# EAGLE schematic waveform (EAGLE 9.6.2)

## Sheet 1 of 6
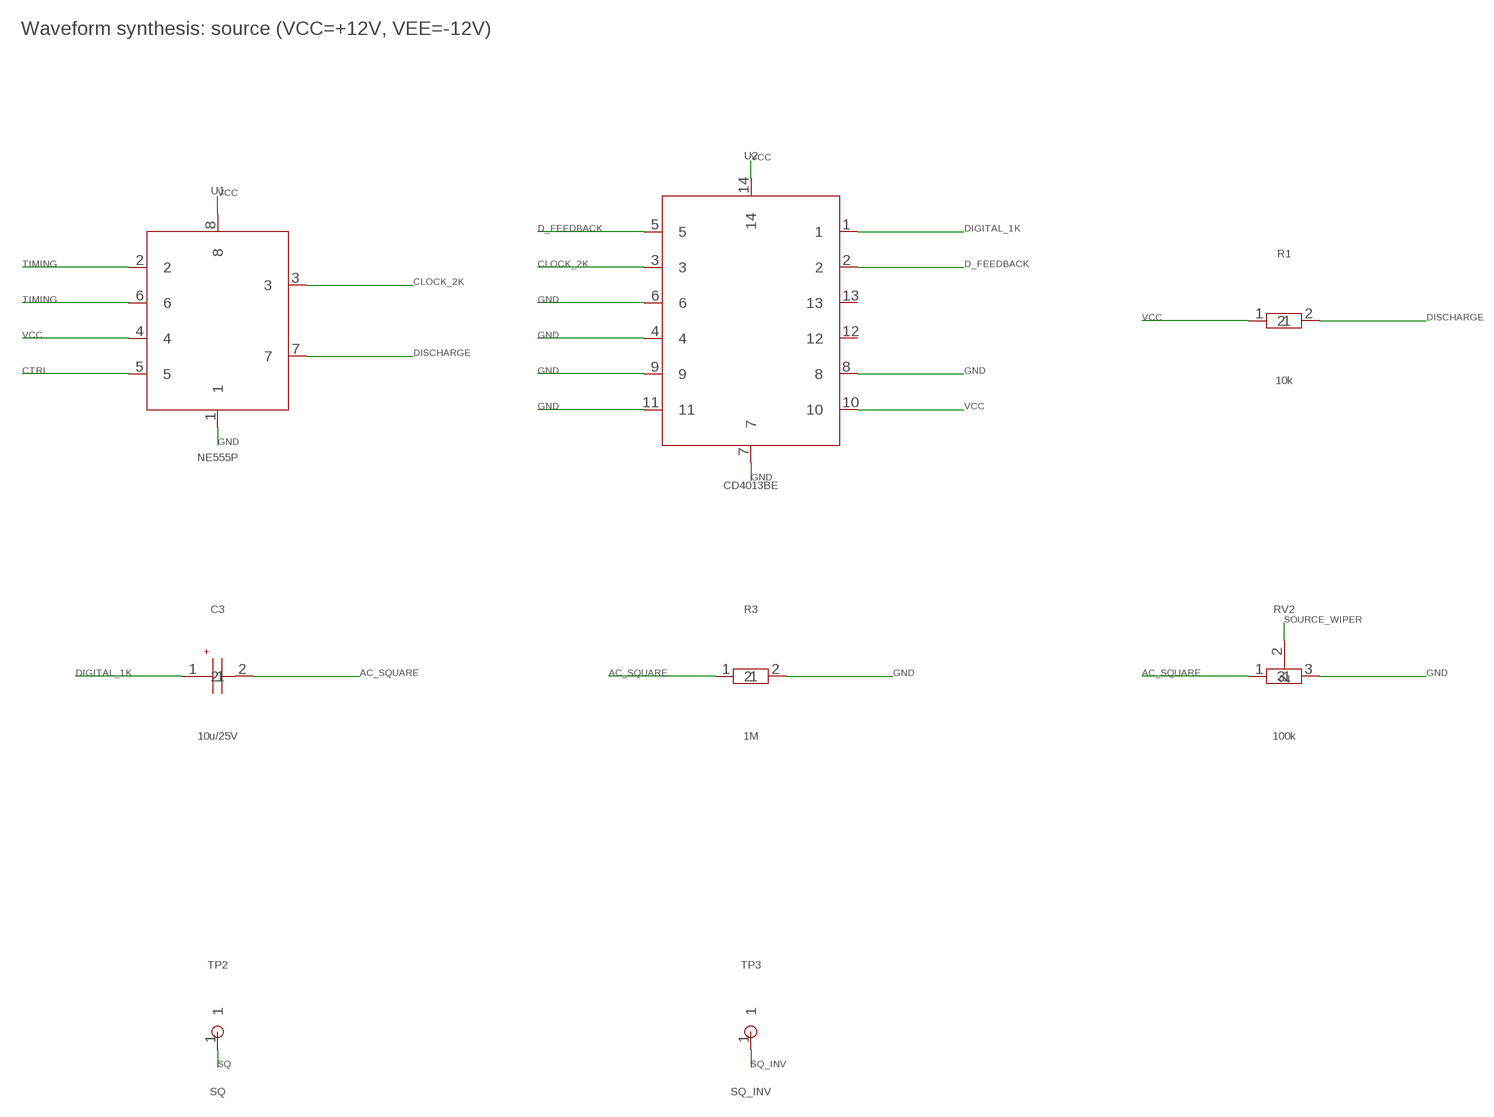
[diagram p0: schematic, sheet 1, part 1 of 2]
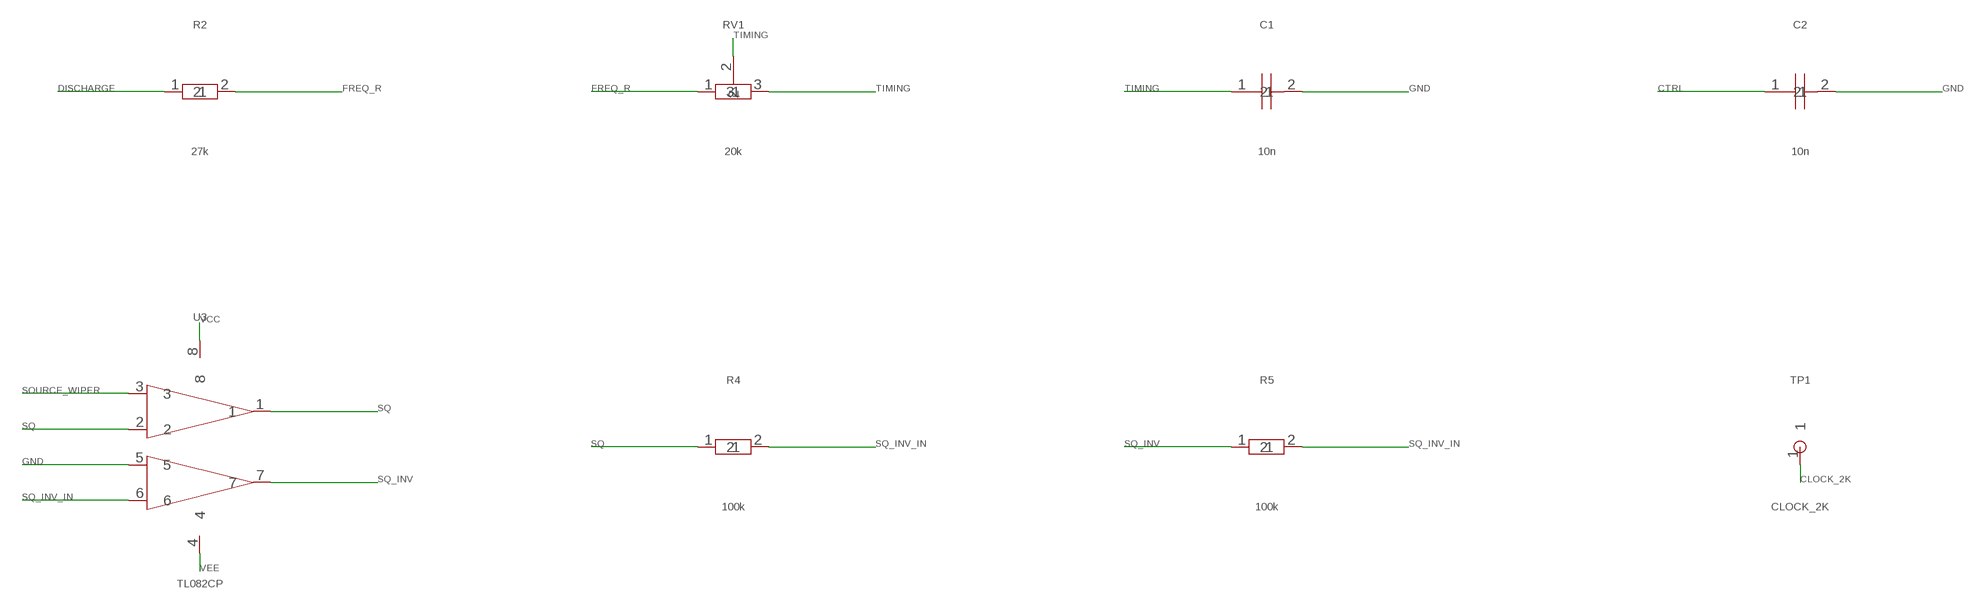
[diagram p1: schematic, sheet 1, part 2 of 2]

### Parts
C1  10n  C  [C_Disc_D5.0mm_W2.5mm_P5.00mm]
C2  10n  C  [C_Disc_D5.0mm_W2.5mm_P5.00mm]
C3  10u/25V  CP  [CP_Radial_D5.0mm_P2.00mm]
R1  10k  R  [R_Axial_DIN0207_L6.3mm_D2.5mm_P7.62mm_Horizontal]
R2  27k  R  [R_Axial_DIN0207_L6.3mm_D2.5mm_P7.62mm_Horizontal]
R3  1M  R  [R_Axial_DIN0207_L6.3mm_D2.5mm_P7.62mm_Horizontal]
R4  100k  R  [R_Axial_DIN0207_L6.3mm_D2.5mm_P7.62mm_Horizontal]
R5  100k  R  [R_Axial_DIN0207_L6.3mm_D2.5mm_P7.62mm_Horizontal]
RV1  20k  POT  [Potentiometer_Bourns_3296W_Vertical]
RV2  100k  POT  [Potentiometer_Bourns_3296W_Vertical]
TP1  CLOCK_2K  TP  [TestPoint_THTPad_D1.5mm_Drill0.7mm]
TP2  SQ  TP  [TestPoint_THTPad_D1.5mm_Drill0.7mm]
TP3  SQ_INV  TP  [TestPoint_THTPad_D1.5mm_Drill0.7mm]
U1  NE555P  NE555  [DIP-8_W7.62mm]
U2  CD4013BE  4013  [DIP-14_W7.62mm]
U3  TL082CP  TL082  [DIP-8_W7.62mm]

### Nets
AC_SQUARE: C3.2 R3.1 RV2.1
CLOCK_2K: TP1.1 U1.3 U2.3
CTRL: C2.1 U1.5
D_FEEDBACK: U2.2 U2.5
DIGITAL_1K: C3.1 U2.1
DISCHARGE: R1.2 R2.1 U1.7
FREQ_R: R2.2 RV1.1
GND: C1.2 C2.2 R3.2 RV2.3 U1.1 U2.4 U2.6 U2.7 U2.8 U2.9 U2.11 U3.5 ; also sheet 2,3,4,5,6
SOURCE_WIPER: RV2.2 U3.3
SQ: R4.1 TP2.1 U3.1 U3.2 ; also sheet 2,3,4,5
SQ_INV: R5.1 TP3.1 U3.7
SQ_INV_IN: R4.2 R5.2 U3.6
TIMING: C1.1 RV1.2 RV1.3 U1.2 U1.6
VCC: R1.1 U1.4 U1.8 U2.10 U2.14 U3.8 ; also sheet 2,3,4,5,6
VEE: U3.4 ; also sheet 2,3,4,5,6
Unconnected: U2.12 U2.13

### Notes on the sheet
- Waveform synthesis: source (VCC=+12V, VEE=-12V)

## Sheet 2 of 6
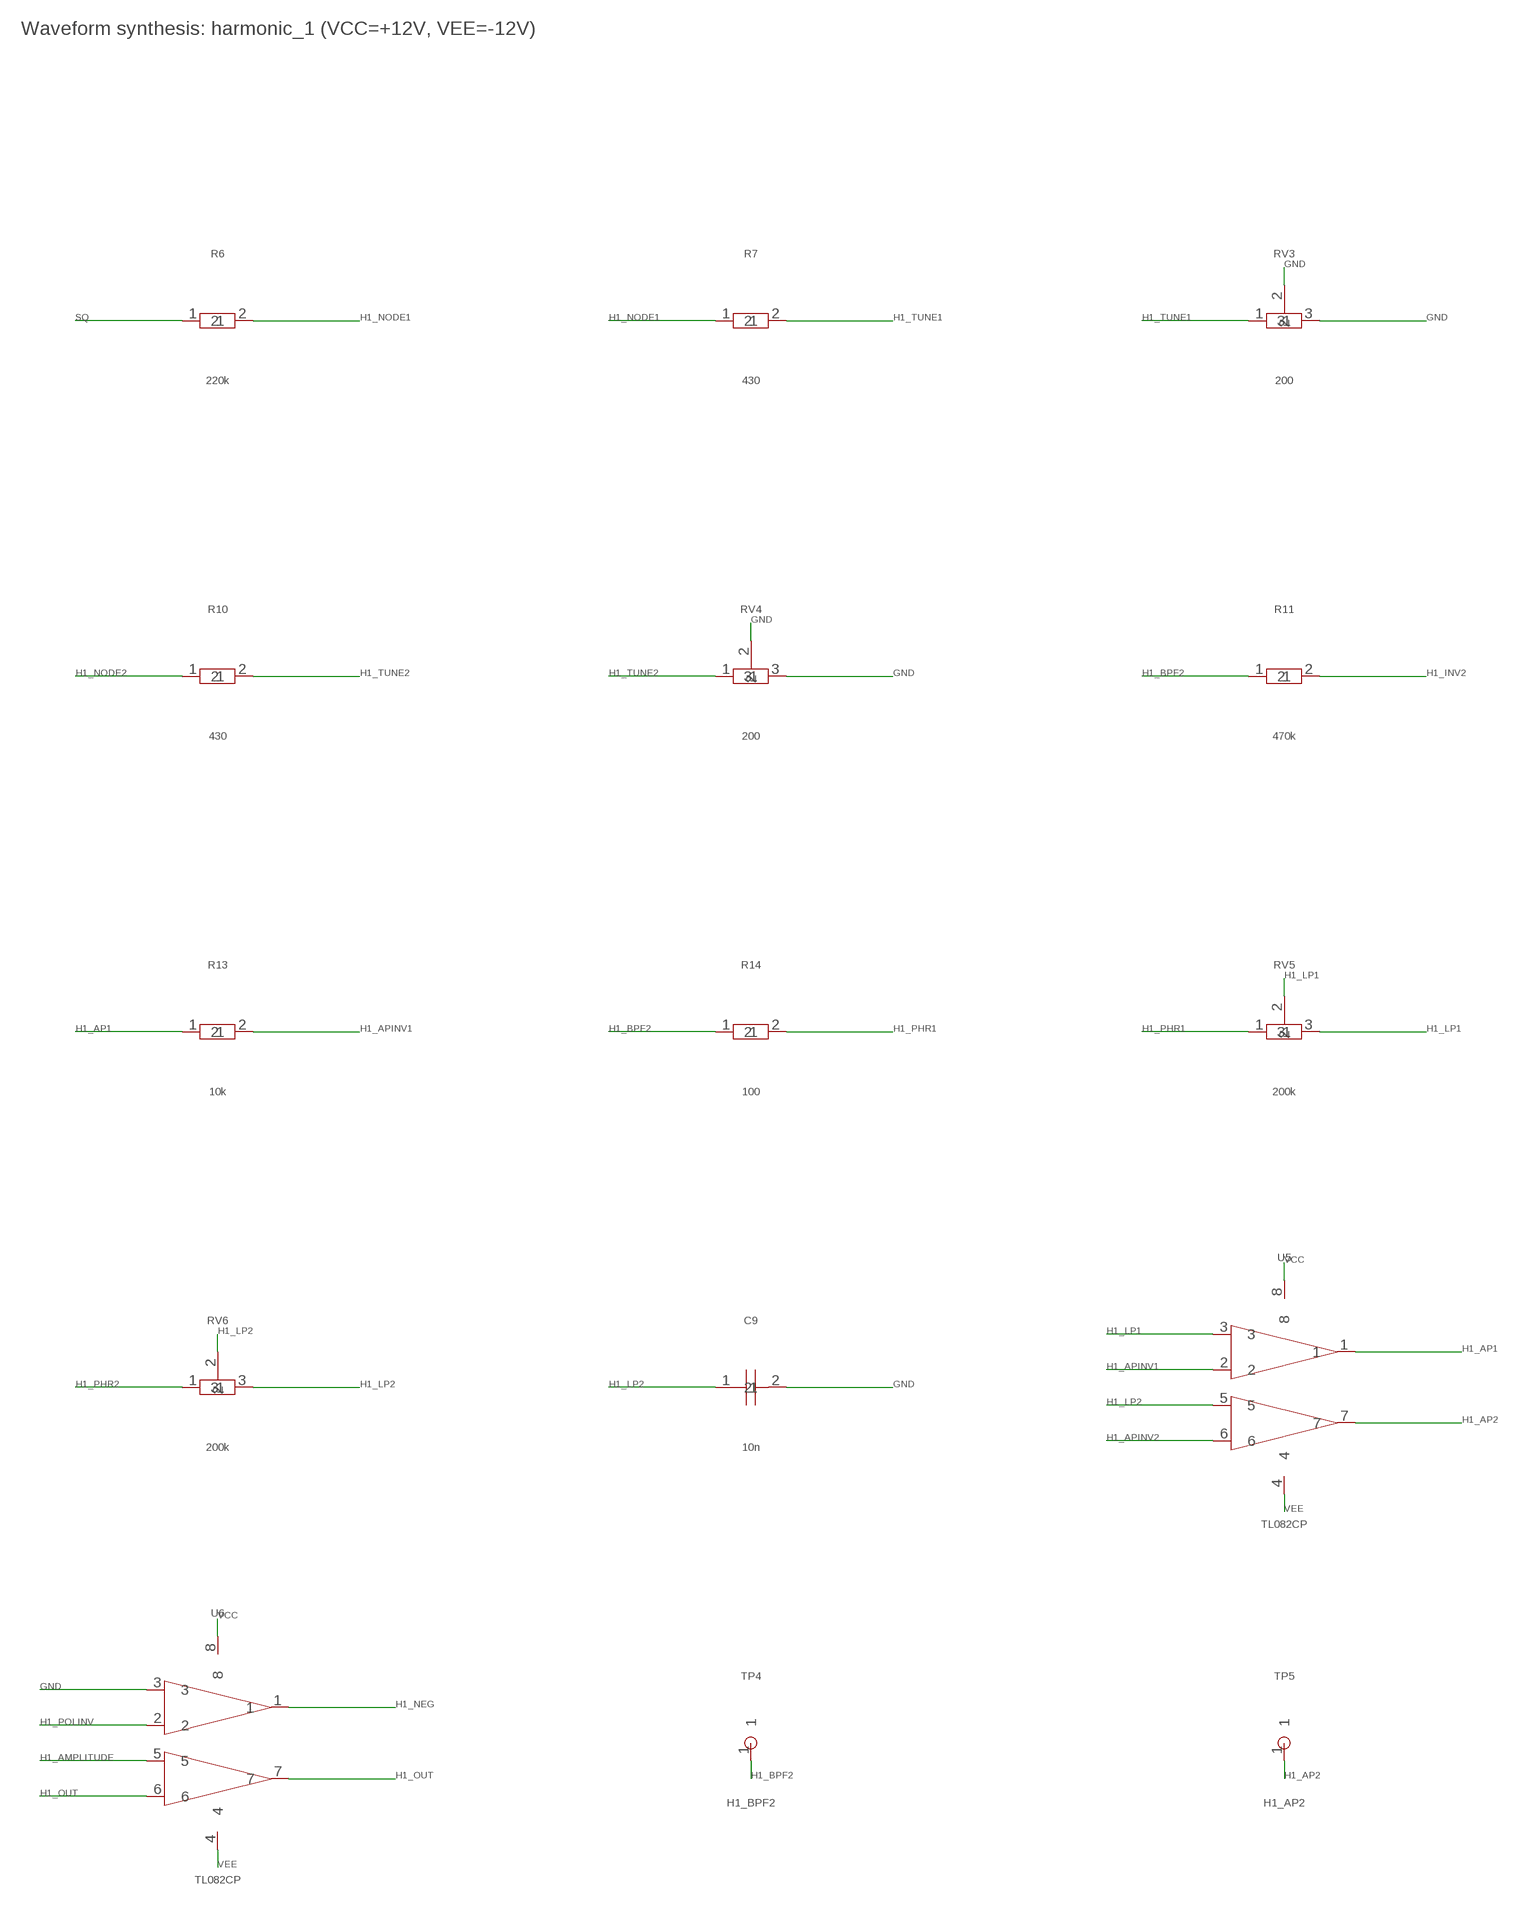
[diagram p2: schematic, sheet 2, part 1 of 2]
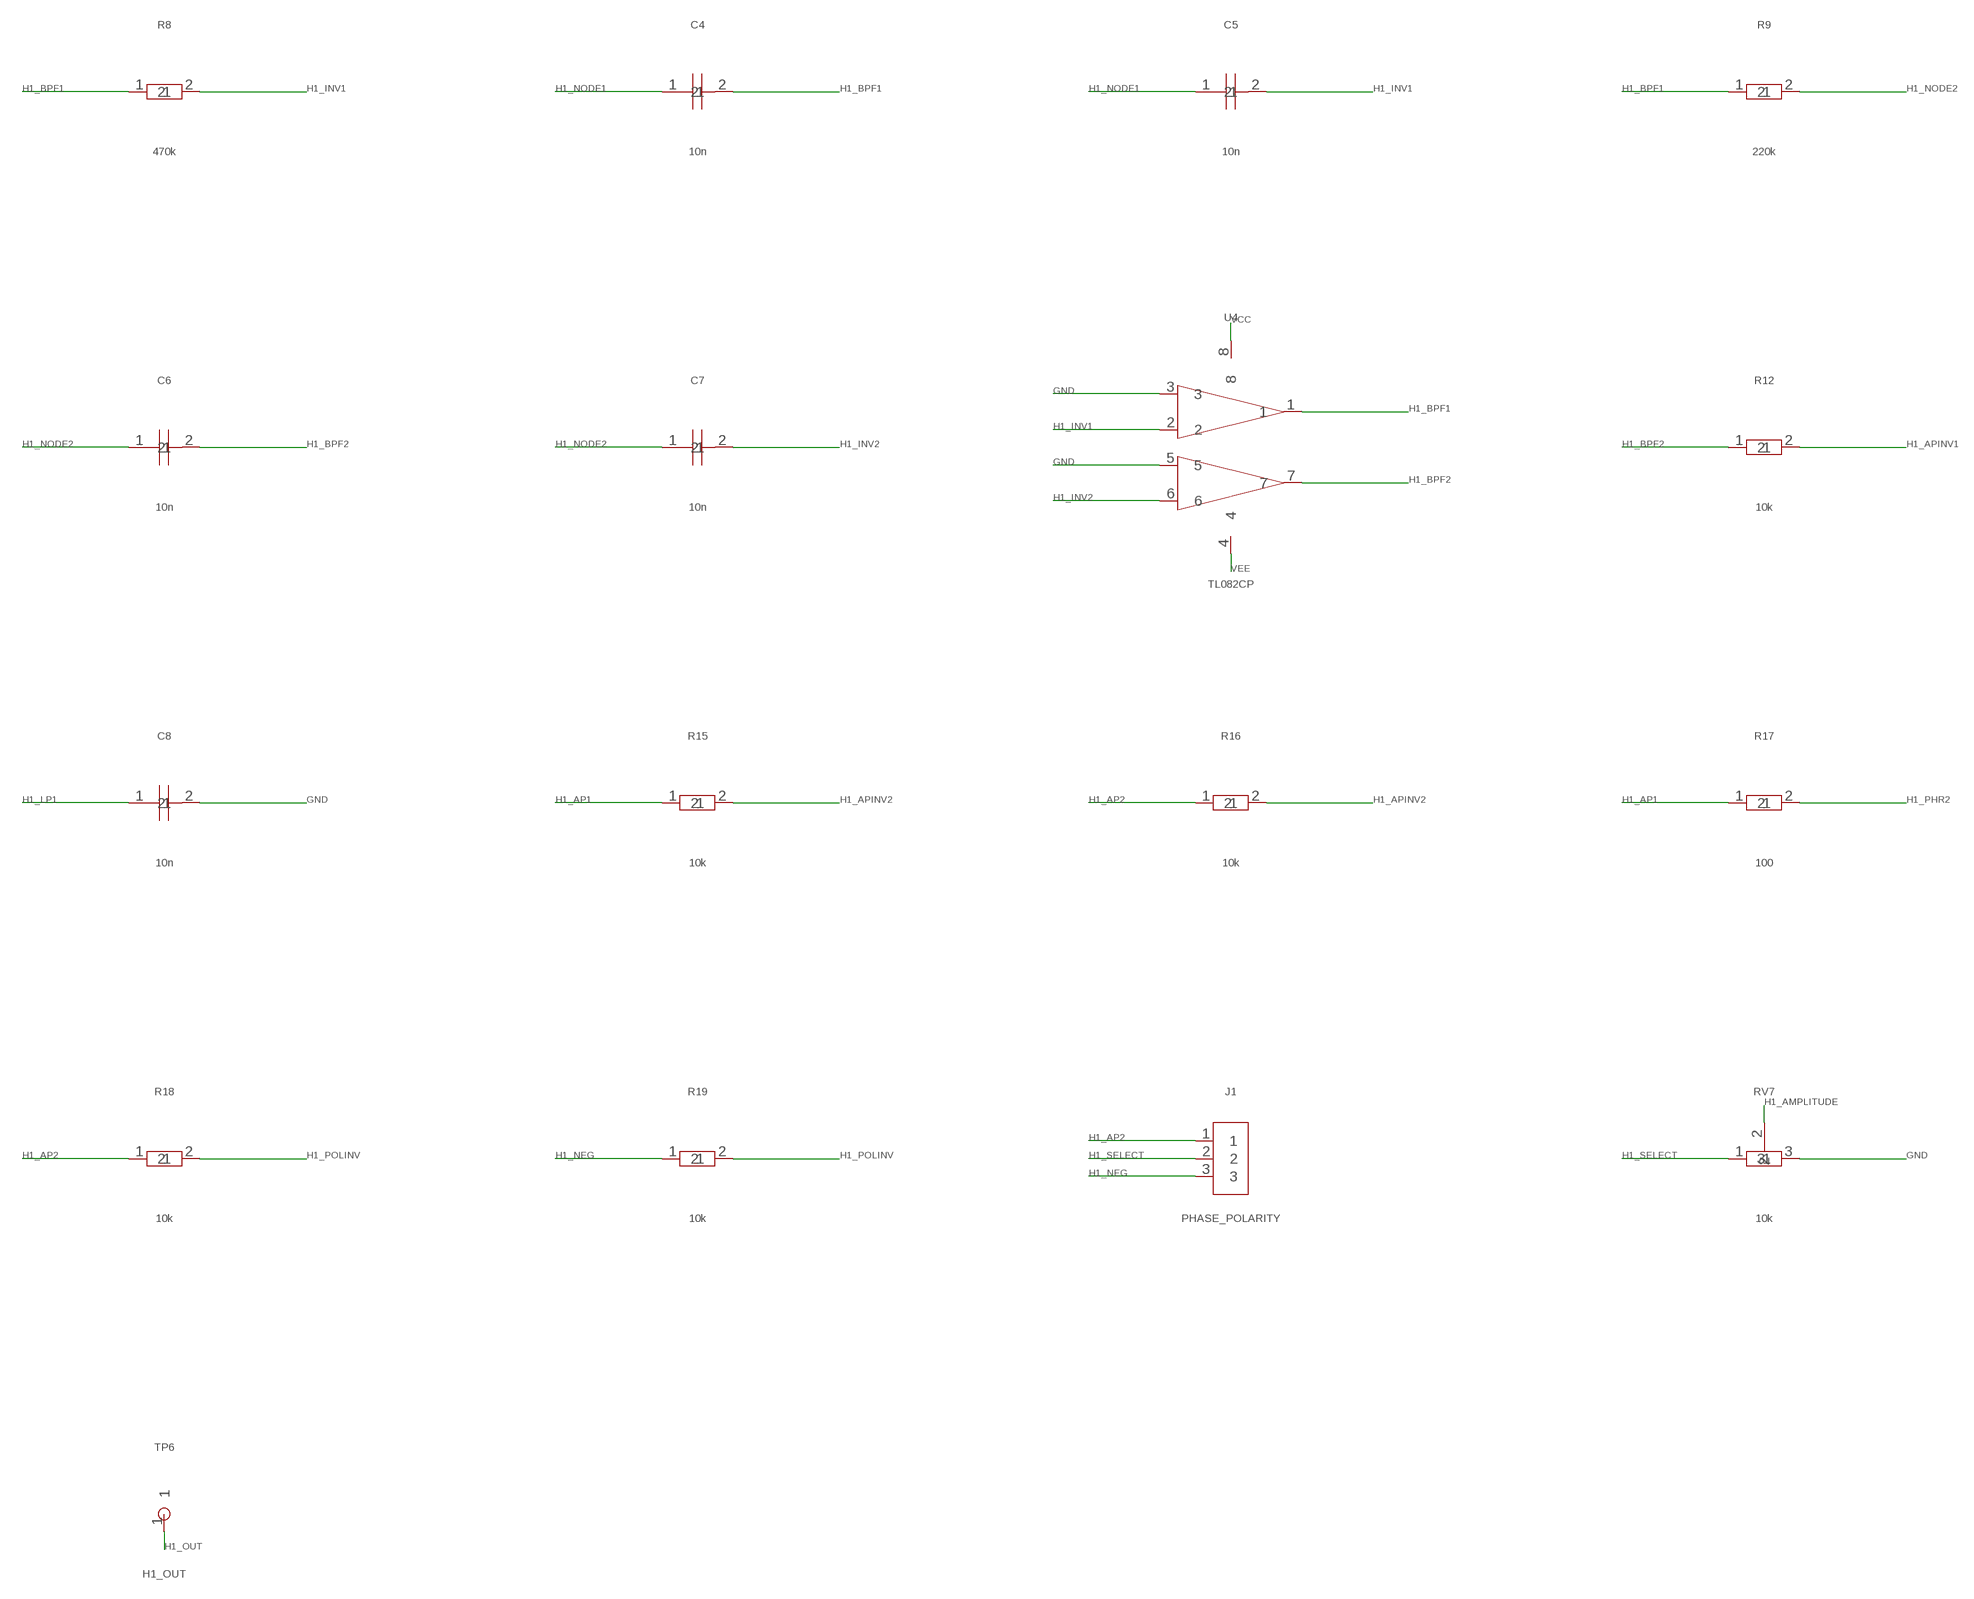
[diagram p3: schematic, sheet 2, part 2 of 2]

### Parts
C4  10n  C  [C_Disc_D5.0mm_W2.5mm_P5.00mm]
C5  10n  C  [C_Disc_D5.0mm_W2.5mm_P5.00mm]
C6  10n  C  [C_Disc_D5.0mm_W2.5mm_P5.00mm]
C7  10n  C  [C_Disc_D5.0mm_W2.5mm_P5.00mm]
C8  10n  C  [C_Disc_D5.0mm_W2.5mm_P5.00mm]
C9  10n  C  [C_Disc_D5.0mm_W2.5mm_P5.00mm]
J1  PHASE_POLARITY  CONN3  [PinHeader_1x03_P2.54mm_Vertical]
R6  220k  R  [R_Axial_DIN0207_L6.3mm_D2.5mm_P7.62mm_Horizontal]
R7  430  R  [R_Axial_DIN0207_L6.3mm_D2.5mm_P7.62mm_Horizontal]
R8  470k  R  [R_Axial_DIN0207_L6.3mm_D2.5mm_P7.62mm_Horizontal]
R9  220k  R  [R_Axial_DIN0207_L6.3mm_D2.5mm_P7.62mm_Horizontal]
R10  430  R  [R_Axial_DIN0207_L6.3mm_D2.5mm_P7.62mm_Horizontal]
R11  470k  R  [R_Axial_DIN0207_L6.3mm_D2.5mm_P7.62mm_Horizontal]
R12  10k  R  [R_Axial_DIN0207_L6.3mm_D2.5mm_P7.62mm_Horizontal]
R13  10k  R  [R_Axial_DIN0207_L6.3mm_D2.5mm_P7.62mm_Horizontal]
R14  100  R  [R_Axial_DIN0207_L6.3mm_D2.5mm_P7.62mm_Horizontal]
R15  10k  R  [R_Axial_DIN0207_L6.3mm_D2.5mm_P7.62mm_Horizontal]
R16  10k  R  [R_Axial_DIN0207_L6.3mm_D2.5mm_P7.62mm_Horizontal]
R17  100  R  [R_Axial_DIN0207_L6.3mm_D2.5mm_P7.62mm_Horizontal]
R18  10k  R  [R_Axial_DIN0207_L6.3mm_D2.5mm_P7.62mm_Horizontal]
R19  10k  R  [R_Axial_DIN0207_L6.3mm_D2.5mm_P7.62mm_Horizontal]
RV3  200  POT  [Potentiometer_Bourns_3296W_Vertical]
RV4  200  POT  [Potentiometer_Bourns_3296W_Vertical]
RV5  200k  POT  [Potentiometer_Bourns_3296W_Vertical]
RV6  200k  POT  [Potentiometer_Bourns_3296W_Vertical]
RV7  10k  POT  [Potentiometer_Bourns_3296W_Vertical]
TP4  H1_BPF2  TP  [TestPoint_THTPad_D1.5mm_Drill0.7mm]
TP5  H1_AP2  TP  [TestPoint_THTPad_D1.5mm_Drill0.7mm]
TP6  H1_OUT  TP  [TestPoint_THTPad_D1.5mm_Drill0.7mm]
U4  TL082CP  TL082  [DIP-8_W7.62mm]
U5  TL082CP  TL082  [DIP-8_W7.62mm]
U6  TL082CP  TL082  [DIP-8_W7.62mm]

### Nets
GND: C8.2 C9.2 RV3.2 RV3.3 RV4.2 RV4.3 RV7.3 U4.3 U4.5 U6.3 ; also sheet 1,3,4,5,6
H1_AMPLITUDE: RV7.2 U6.5
H1_AP1: R13.1 R15.1 R17.1 U5.1
H1_AP2: J1.1 R16.1 R18.1 TP5.1 U5.7
H1_APINV1: R12.2 R13.2 U5.2
H1_APINV2: R15.2 R16.2 U5.6
H1_BPF1: C4.2 R8.1 R9.1 U4.1
H1_BPF2: C6.2 R11.1 R12.1 R14.1 TP4.1 U4.7
H1_INV1: C5.2 R8.2 U4.2
H1_INV2: C7.2 R11.2 U4.6
H1_LP1: C8.1 RV5.2 RV5.3 U5.3
H1_LP2: C9.1 RV6.2 RV6.3 U5.5
H1_NEG: J1.3 R19.1 U6.1
H1_NODE1: C4.1 C5.1 R6.2 R7.1
H1_NODE2: C6.1 C7.1 R9.2 R10.1
H1_OUT: TP6.1 U6.6 U6.7 ; also sheet 6
H1_PHR1: R14.2 RV5.1
H1_PHR2: R17.2 RV6.1
H1_POLINV: R18.2 R19.2 U6.2
H1_SELECT: J1.2 RV7.1
H1_TUNE1: R7.2 RV3.1
H1_TUNE2: R10.2 RV4.1
SQ: R6.1 ; also sheet 1,3,4,5
VCC: U4.8 U5.8 U6.8 ; also sheet 1,3,4,5,6
VEE: U4.4 U5.4 U6.4 ; also sheet 1,3,4,5,6

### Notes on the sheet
- Waveform synthesis: harmonic_1 (VCC=+12V, VEE=-12V)

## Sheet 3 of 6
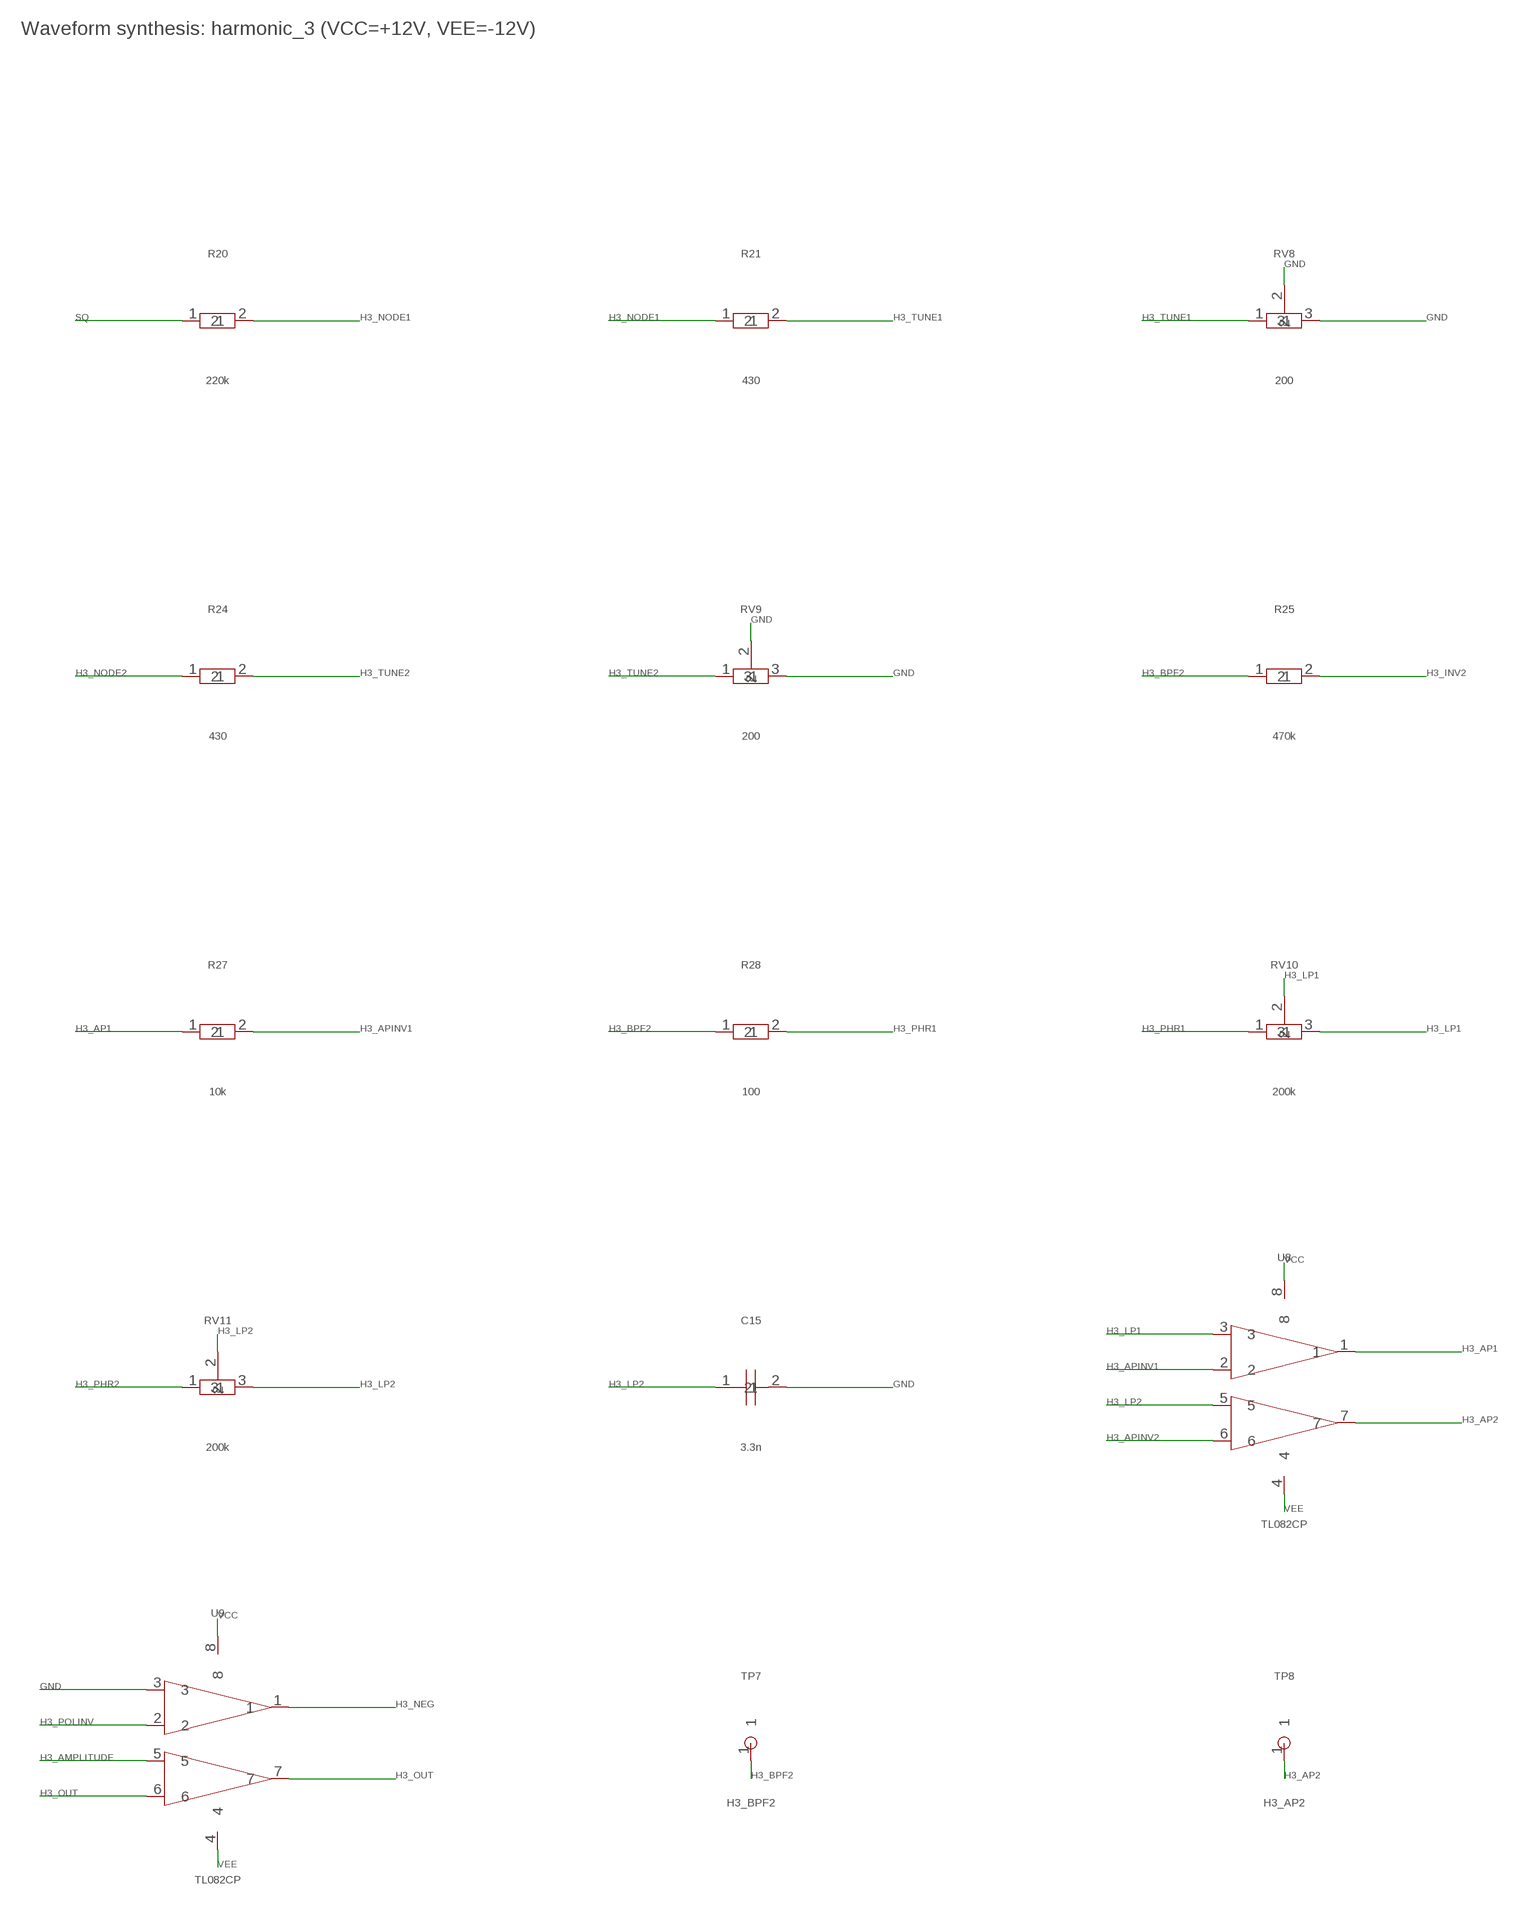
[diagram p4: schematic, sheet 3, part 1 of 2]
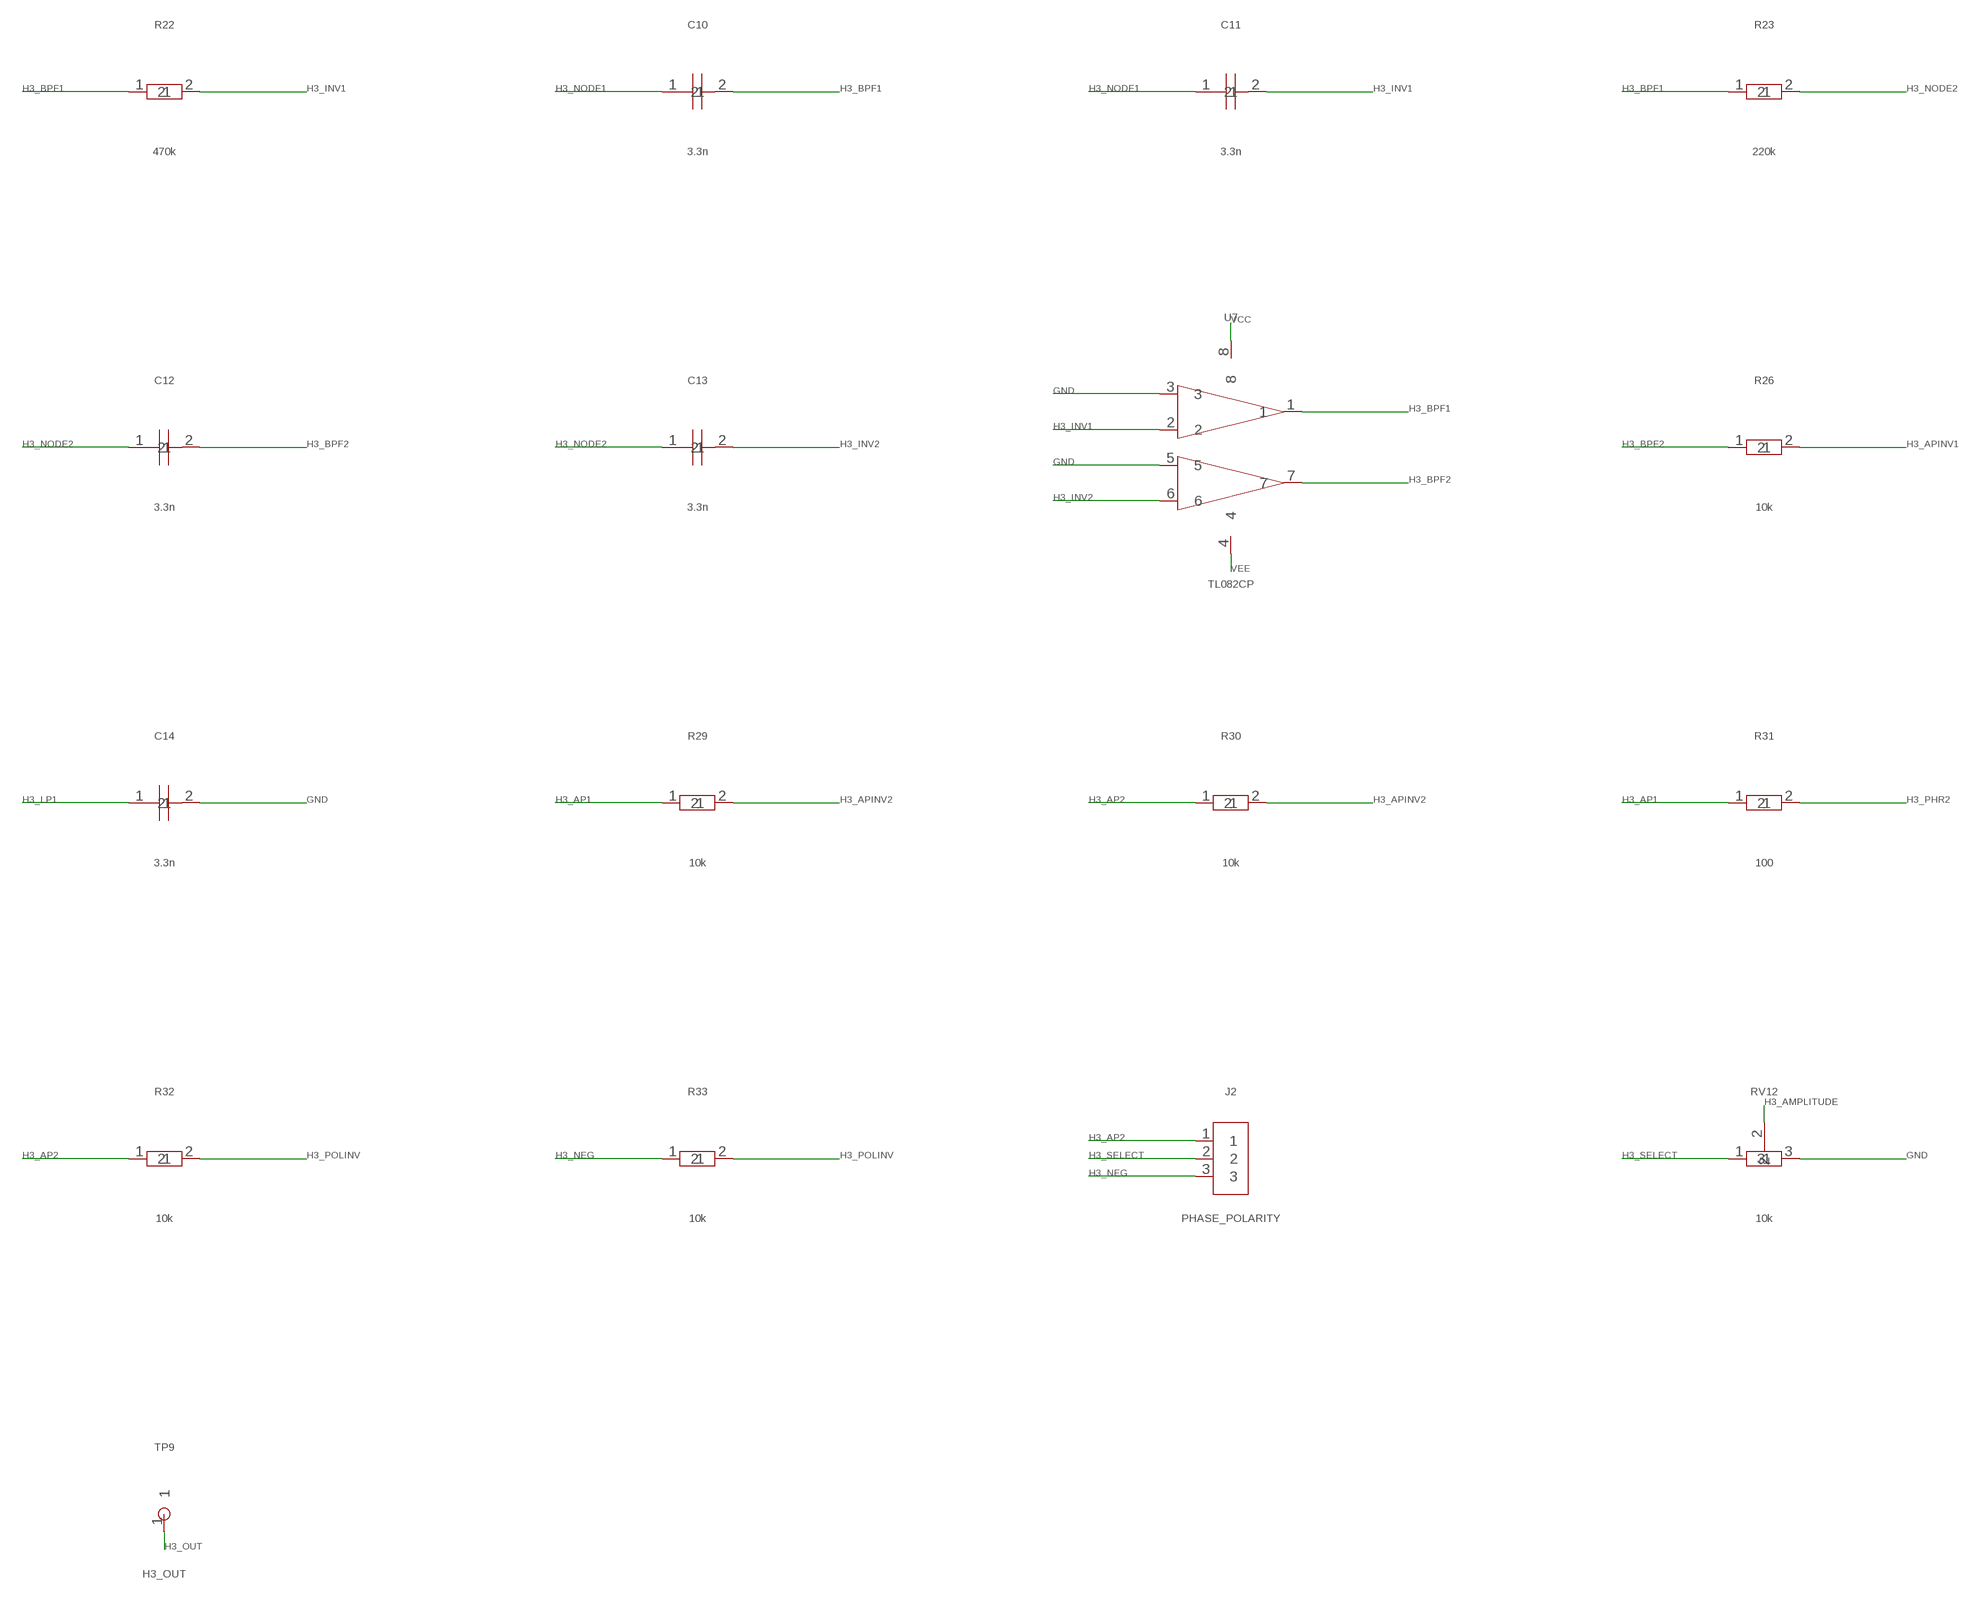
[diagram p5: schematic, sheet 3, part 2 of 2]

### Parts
C10  3.3n  C  [C_Disc_D5.0mm_W2.5mm_P5.00mm]
C11  3.3n  C  [C_Disc_D5.0mm_W2.5mm_P5.00mm]
C12  3.3n  C  [C_Disc_D5.0mm_W2.5mm_P5.00mm]
C13  3.3n  C  [C_Disc_D5.0mm_W2.5mm_P5.00mm]
C14  3.3n  C  [C_Disc_D5.0mm_W2.5mm_P5.00mm]
C15  3.3n  C  [C_Disc_D5.0mm_W2.5mm_P5.00mm]
J2  PHASE_POLARITY  CONN3  [PinHeader_1x03_P2.54mm_Vertical]
R20  220k  R  [R_Axial_DIN0207_L6.3mm_D2.5mm_P7.62mm_Horizontal]
R21  430  R  [R_Axial_DIN0207_L6.3mm_D2.5mm_P7.62mm_Horizontal]
R22  470k  R  [R_Axial_DIN0207_L6.3mm_D2.5mm_P7.62mm_Horizontal]
R23  220k  R  [R_Axial_DIN0207_L6.3mm_D2.5mm_P7.62mm_Horizontal]
R24  430  R  [R_Axial_DIN0207_L6.3mm_D2.5mm_P7.62mm_Horizontal]
R25  470k  R  [R_Axial_DIN0207_L6.3mm_D2.5mm_P7.62mm_Horizontal]
R26  10k  R  [R_Axial_DIN0207_L6.3mm_D2.5mm_P7.62mm_Horizontal]
R27  10k  R  [R_Axial_DIN0207_L6.3mm_D2.5mm_P7.62mm_Horizontal]
R28  100  R  [R_Axial_DIN0207_L6.3mm_D2.5mm_P7.62mm_Horizontal]
R29  10k  R  [R_Axial_DIN0207_L6.3mm_D2.5mm_P7.62mm_Horizontal]
R30  10k  R  [R_Axial_DIN0207_L6.3mm_D2.5mm_P7.62mm_Horizontal]
R31  100  R  [R_Axial_DIN0207_L6.3mm_D2.5mm_P7.62mm_Horizontal]
R32  10k  R  [R_Axial_DIN0207_L6.3mm_D2.5mm_P7.62mm_Horizontal]
R33  10k  R  [R_Axial_DIN0207_L6.3mm_D2.5mm_P7.62mm_Horizontal]
RV8  200  POT  [Potentiometer_Bourns_3296W_Vertical]
RV9  200  POT  [Potentiometer_Bourns_3296W_Vertical]
RV10  200k  POT  [Potentiometer_Bourns_3296W_Vertical]
RV11  200k  POT  [Potentiometer_Bourns_3296W_Vertical]
RV12  10k  POT  [Potentiometer_Bourns_3296W_Vertical]
TP7  H3_BPF2  TP  [TestPoint_THTPad_D1.5mm_Drill0.7mm]
TP8  H3_AP2  TP  [TestPoint_THTPad_D1.5mm_Drill0.7mm]
TP9  H3_OUT  TP  [TestPoint_THTPad_D1.5mm_Drill0.7mm]
U7  TL082CP  TL082  [DIP-8_W7.62mm]
U8  TL082CP  TL082  [DIP-8_W7.62mm]
U9  TL082CP  TL082  [DIP-8_W7.62mm]

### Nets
GND: C14.2 C15.2 RV8.2 RV8.3 RV9.2 RV9.3 RV12.3 U7.3 U7.5 U9.3 ; also sheet 1,2,4,5,6
H3_AMPLITUDE: RV12.2 U9.5
H3_AP1: R27.1 R29.1 R31.1 U8.1
H3_AP2: J2.1 R30.1 R32.1 TP8.1 U8.7
H3_APINV1: R26.2 R27.2 U8.2
H3_APINV2: R29.2 R30.2 U8.6
H3_BPF1: C10.2 R22.1 R23.1 U7.1
H3_BPF2: C12.2 R25.1 R26.1 R28.1 TP7.1 U7.7
H3_INV1: C11.2 R22.2 U7.2
H3_INV2: C13.2 R25.2 U7.6
H3_LP1: C14.1 RV10.2 RV10.3 U8.3
H3_LP2: C15.1 RV11.2 RV11.3 U8.5
H3_NEG: J2.3 R33.1 U9.1
H3_NODE1: C10.1 C11.1 R20.2 R21.1
H3_NODE2: C12.1 C13.1 R23.2 R24.1
H3_OUT: TP9.1 U9.6 U9.7 ; also sheet 6
H3_PHR1: R28.2 RV10.1
H3_PHR2: R31.2 RV11.1
H3_POLINV: R32.2 R33.2 U9.2
H3_SELECT: J2.2 RV12.1
H3_TUNE1: R21.2 RV8.1
H3_TUNE2: R24.2 RV9.1
SQ: R20.1 ; also sheet 1,2,4,5
VCC: U7.8 U8.8 U9.8 ; also sheet 1,2,4,5,6
VEE: U7.4 U8.4 U9.4 ; also sheet 1,2,4,5,6

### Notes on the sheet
- Waveform synthesis: harmonic_3 (VCC=+12V, VEE=-12V)

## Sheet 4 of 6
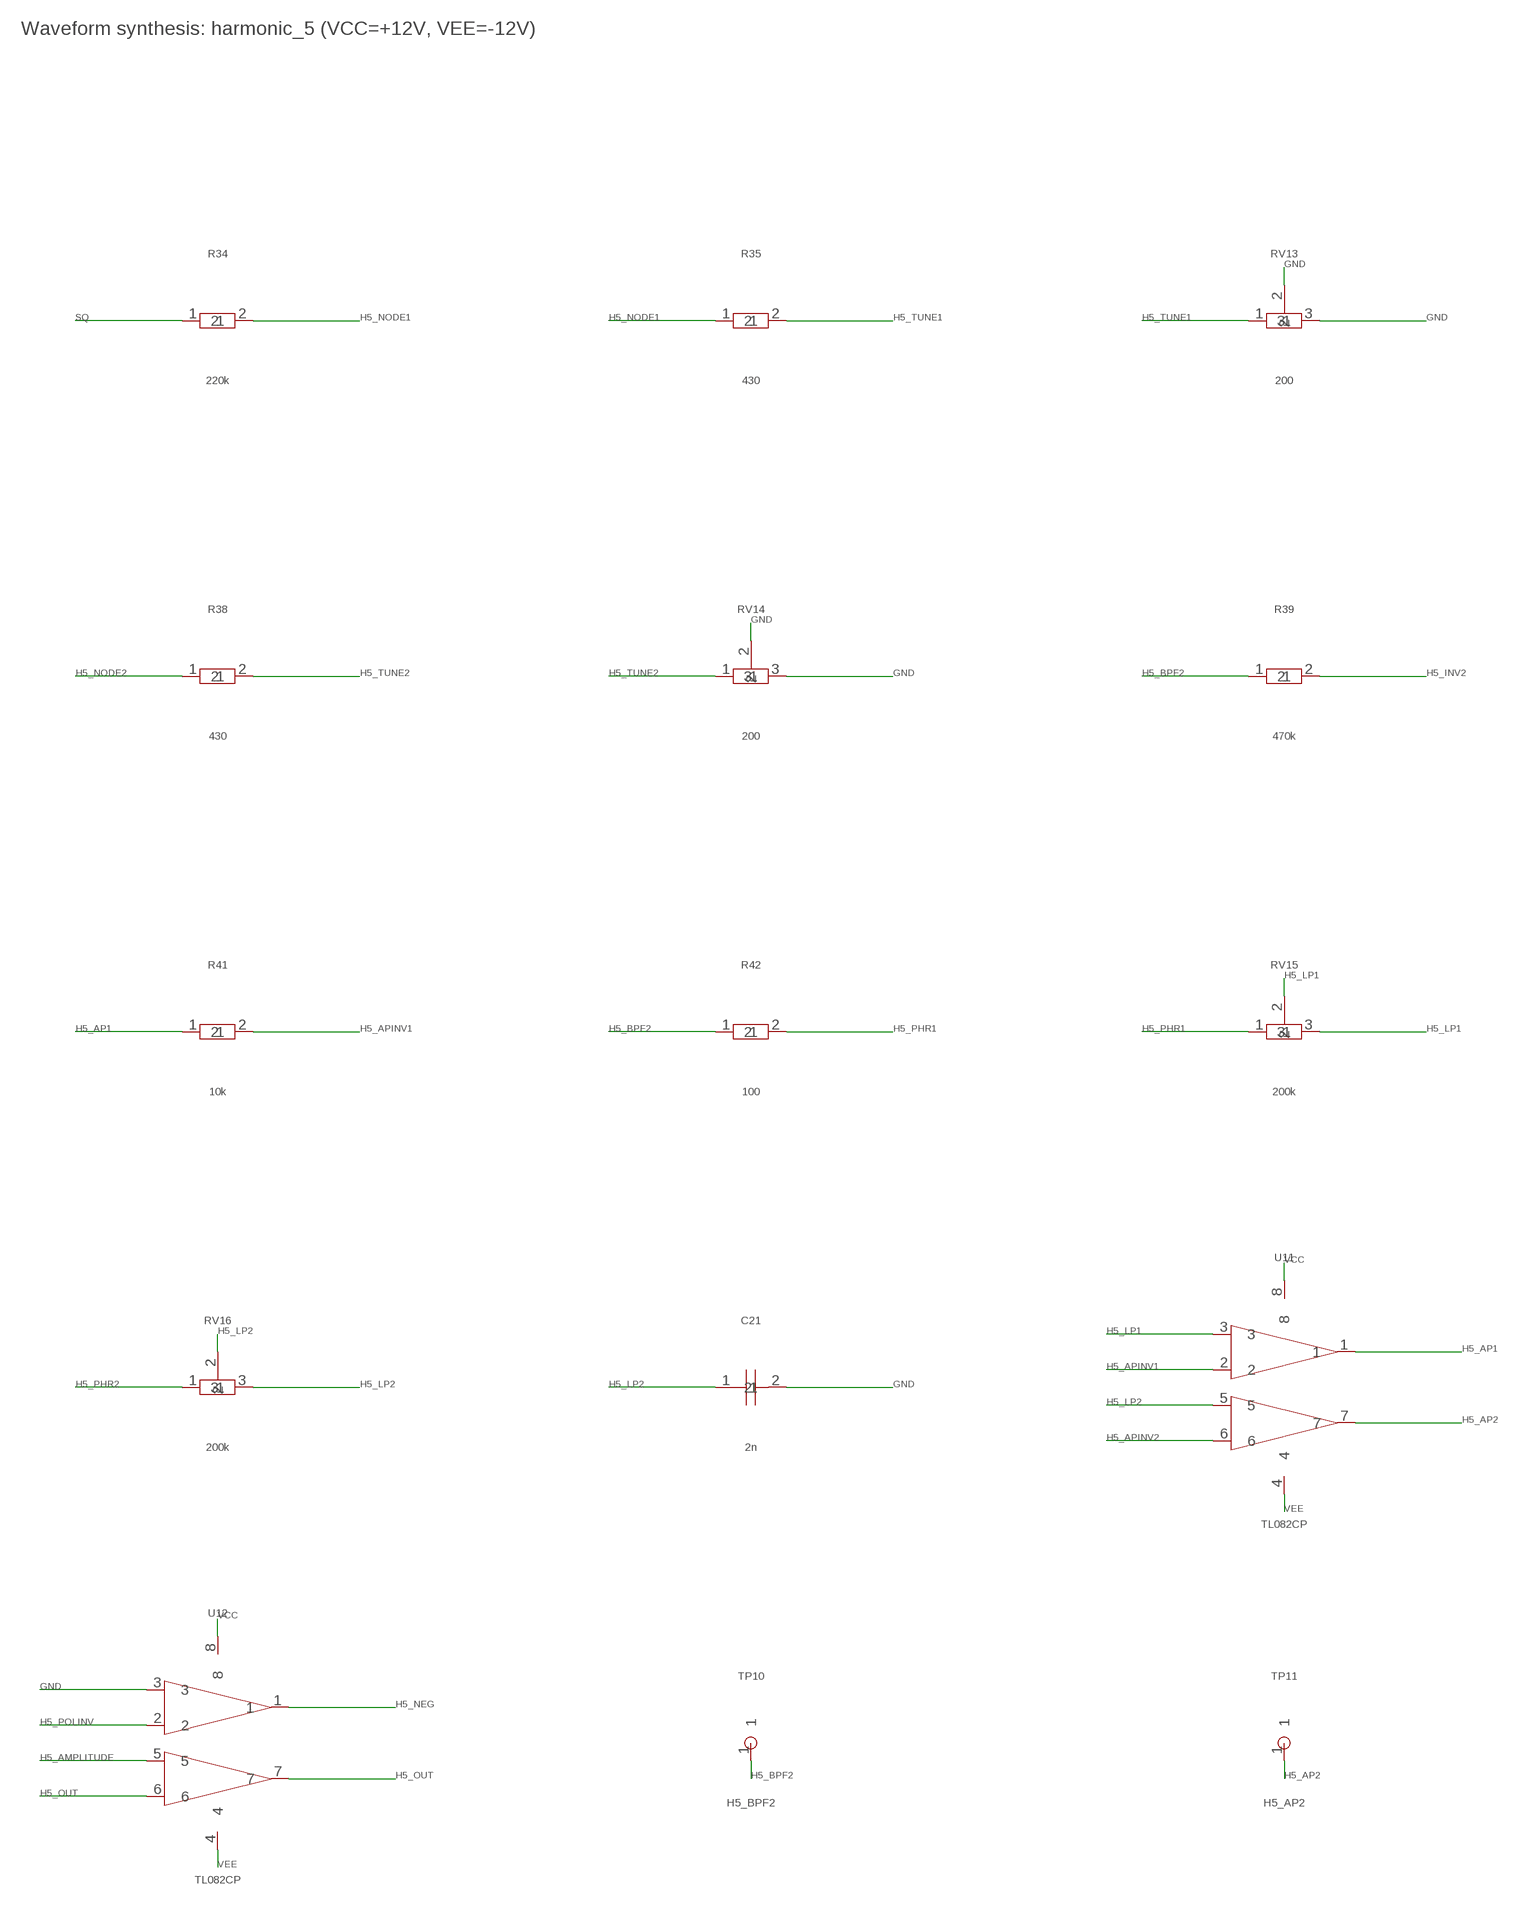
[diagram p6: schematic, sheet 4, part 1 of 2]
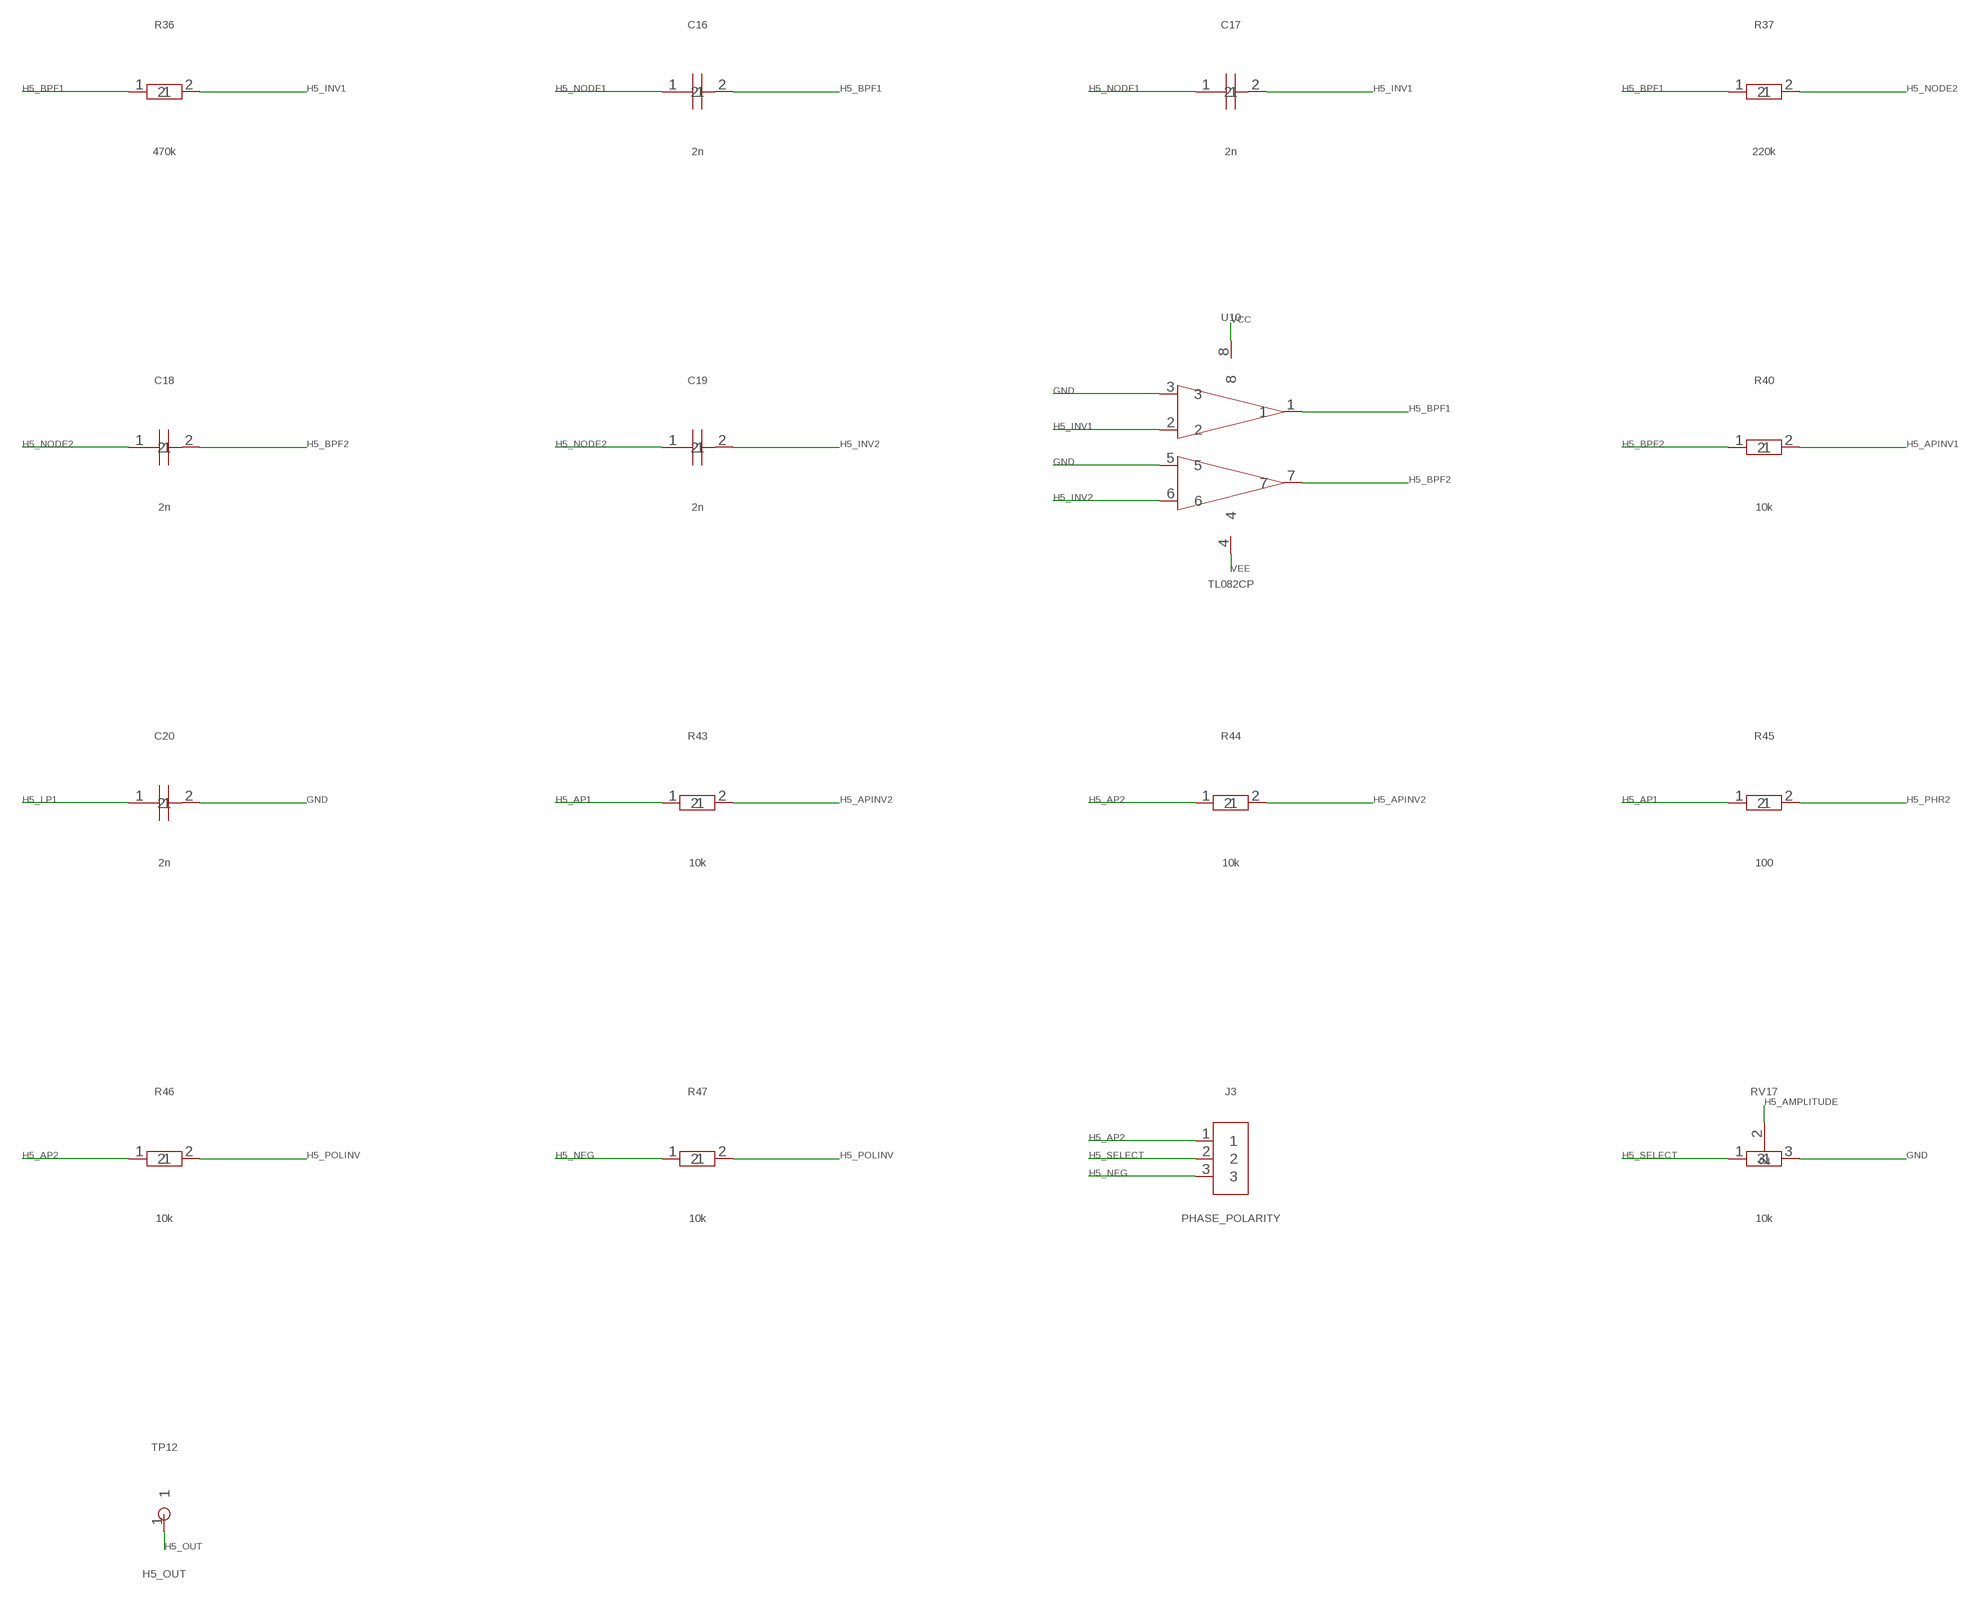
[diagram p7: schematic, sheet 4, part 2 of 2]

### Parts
C16  2n  C  [C_Disc_D5.0mm_W2.5mm_P5.00mm]
C17  2n  C  [C_Disc_D5.0mm_W2.5mm_P5.00mm]
C18  2n  C  [C_Disc_D5.0mm_W2.5mm_P5.00mm]
C19  2n  C  [C_Disc_D5.0mm_W2.5mm_P5.00mm]
C20  2n  C  [C_Disc_D5.0mm_W2.5mm_P5.00mm]
C21  2n  C  [C_Disc_D5.0mm_W2.5mm_P5.00mm]
J3  PHASE_POLARITY  CONN3  [PinHeader_1x03_P2.54mm_Vertical]
R34  220k  R  [R_Axial_DIN0207_L6.3mm_D2.5mm_P7.62mm_Horizontal]
R35  430  R  [R_Axial_DIN0207_L6.3mm_D2.5mm_P7.62mm_Horizontal]
R36  470k  R  [R_Axial_DIN0207_L6.3mm_D2.5mm_P7.62mm_Horizontal]
R37  220k  R  [R_Axial_DIN0207_L6.3mm_D2.5mm_P7.62mm_Horizontal]
R38  430  R  [R_Axial_DIN0207_L6.3mm_D2.5mm_P7.62mm_Horizontal]
R39  470k  R  [R_Axial_DIN0207_L6.3mm_D2.5mm_P7.62mm_Horizontal]
R40  10k  R  [R_Axial_DIN0207_L6.3mm_D2.5mm_P7.62mm_Horizontal]
R41  10k  R  [R_Axial_DIN0207_L6.3mm_D2.5mm_P7.62mm_Horizontal]
R42  100  R  [R_Axial_DIN0207_L6.3mm_D2.5mm_P7.62mm_Horizontal]
R43  10k  R  [R_Axial_DIN0207_L6.3mm_D2.5mm_P7.62mm_Horizontal]
R44  10k  R  [R_Axial_DIN0207_L6.3mm_D2.5mm_P7.62mm_Horizontal]
R45  100  R  [R_Axial_DIN0207_L6.3mm_D2.5mm_P7.62mm_Horizontal]
R46  10k  R  [R_Axial_DIN0207_L6.3mm_D2.5mm_P7.62mm_Horizontal]
R47  10k  R  [R_Axial_DIN0207_L6.3mm_D2.5mm_P7.62mm_Horizontal]
RV13  200  POT  [Potentiometer_Bourns_3296W_Vertical]
RV14  200  POT  [Potentiometer_Bourns_3296W_Vertical]
RV15  200k  POT  [Potentiometer_Bourns_3296W_Vertical]
RV16  200k  POT  [Potentiometer_Bourns_3296W_Vertical]
RV17  10k  POT  [Potentiometer_Bourns_3296W_Vertical]
TP10  H5_BPF2  TP  [TestPoint_THTPad_D1.5mm_Drill0.7mm]
TP11  H5_AP2  TP  [TestPoint_THTPad_D1.5mm_Drill0.7mm]
TP12  H5_OUT  TP  [TestPoint_THTPad_D1.5mm_Drill0.7mm]
U10  TL082CP  TL082  [DIP-8_W7.62mm]
U11  TL082CP  TL082  [DIP-8_W7.62mm]
U12  TL082CP  TL082  [DIP-8_W7.62mm]

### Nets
GND: C20.2 C21.2 RV13.2 RV13.3 RV14.2 RV14.3 RV17.3 U10.3 U10.5 U12.3 ; also sheet 1,2,3,5,6
H5_AMPLITUDE: RV17.2 U12.5
H5_AP1: R41.1 R43.1 R45.1 U11.1
H5_AP2: J3.1 R44.1 R46.1 TP11.1 U11.7
H5_APINV1: R40.2 R41.2 U11.2
H5_APINV2: R43.2 R44.2 U11.6
H5_BPF1: C16.2 R36.1 R37.1 U10.1
H5_BPF2: C18.2 R39.1 R40.1 R42.1 TP10.1 U10.7
H5_INV1: C17.2 R36.2 U10.2
H5_INV2: C19.2 R39.2 U10.6
H5_LP1: C20.1 RV15.2 RV15.3 U11.3
H5_LP2: C21.1 RV16.2 RV16.3 U11.5
H5_NEG: J3.3 R47.1 U12.1
H5_NODE1: C16.1 C17.1 R34.2 R35.1
H5_NODE2: C18.1 C19.1 R37.2 R38.1
H5_OUT: TP12.1 U12.6 U12.7 ; also sheet 6
H5_PHR1: R42.2 RV15.1
H5_PHR2: R45.2 RV16.1
H5_POLINV: R46.2 R47.2 U12.2
H5_SELECT: J3.2 RV17.1
H5_TUNE1: R35.2 RV13.1
H5_TUNE2: R38.2 RV14.1
SQ: R34.1 ; also sheet 1,2,3,5
VCC: U10.8 U11.8 U12.8 ; also sheet 1,2,3,5,6
VEE: U10.4 U11.4 U12.4 ; also sheet 1,2,3,5,6

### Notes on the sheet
- Waveform synthesis: harmonic_5 (VCC=+12V, VEE=-12V)

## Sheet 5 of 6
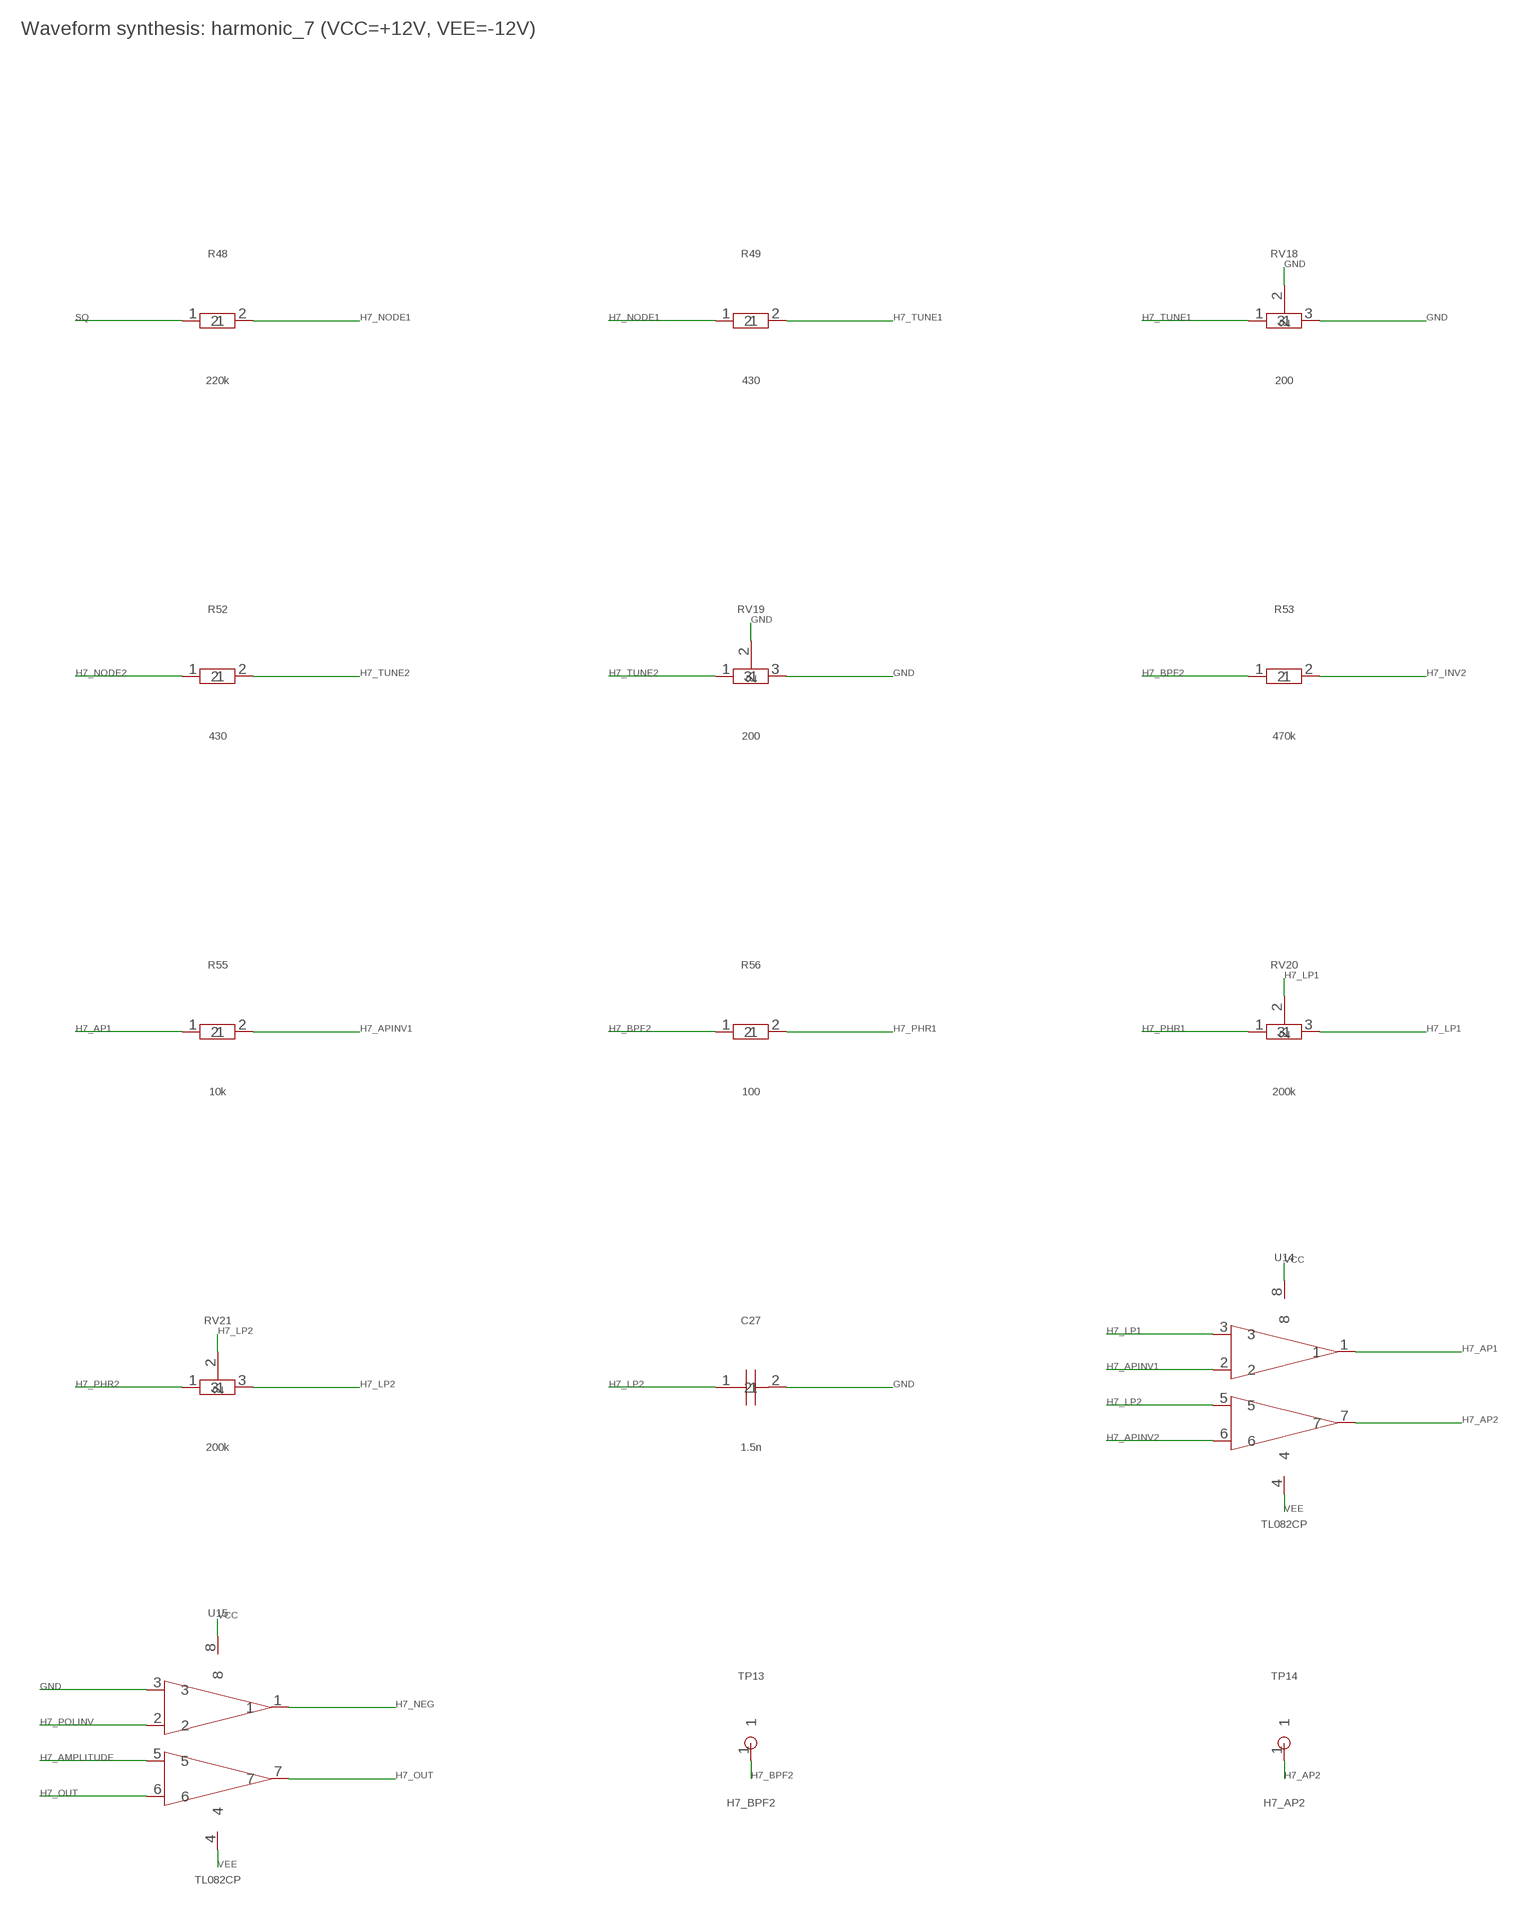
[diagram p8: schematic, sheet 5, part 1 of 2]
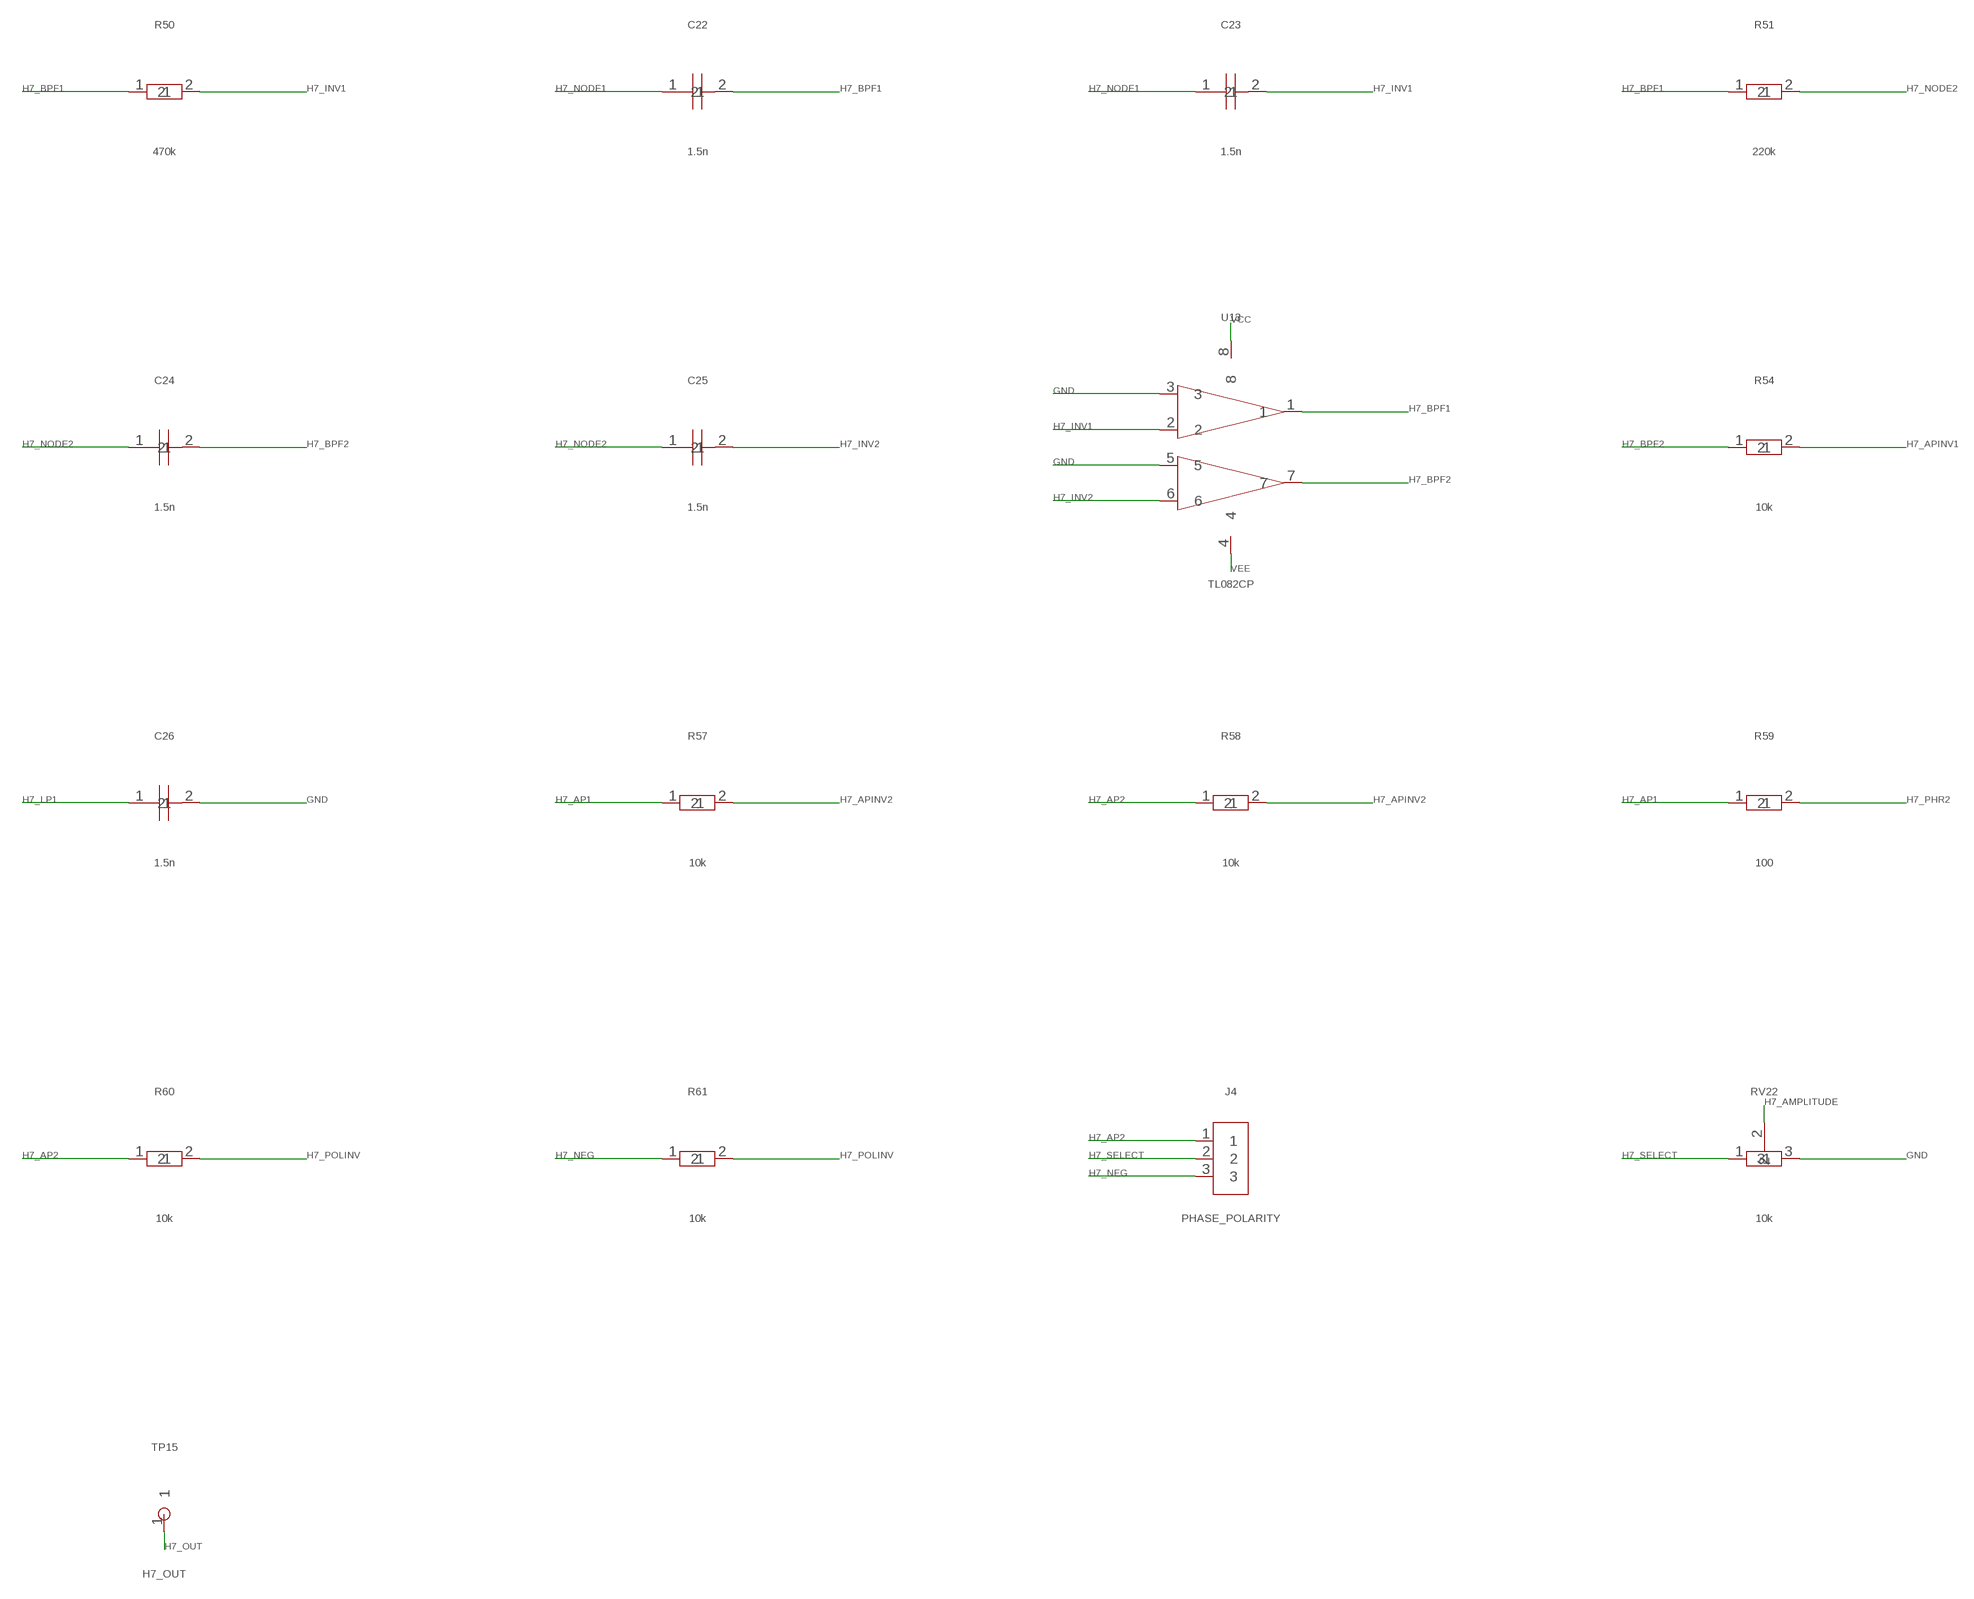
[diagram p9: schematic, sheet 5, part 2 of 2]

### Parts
C22  1.5n  C  [C_Disc_D5.0mm_W2.5mm_P5.00mm]
C23  1.5n  C  [C_Disc_D5.0mm_W2.5mm_P5.00mm]
C24  1.5n  C  [C_Disc_D5.0mm_W2.5mm_P5.00mm]
C25  1.5n  C  [C_Disc_D5.0mm_W2.5mm_P5.00mm]
C26  1.5n  C  [C_Disc_D5.0mm_W2.5mm_P5.00mm]
C27  1.5n  C  [C_Disc_D5.0mm_W2.5mm_P5.00mm]
J4  PHASE_POLARITY  CONN3  [PinHeader_1x03_P2.54mm_Vertical]
R48  220k  R  [R_Axial_DIN0207_L6.3mm_D2.5mm_P7.62mm_Horizontal]
R49  430  R  [R_Axial_DIN0207_L6.3mm_D2.5mm_P7.62mm_Horizontal]
R50  470k  R  [R_Axial_DIN0207_L6.3mm_D2.5mm_P7.62mm_Horizontal]
R51  220k  R  [R_Axial_DIN0207_L6.3mm_D2.5mm_P7.62mm_Horizontal]
R52  430  R  [R_Axial_DIN0207_L6.3mm_D2.5mm_P7.62mm_Horizontal]
R53  470k  R  [R_Axial_DIN0207_L6.3mm_D2.5mm_P7.62mm_Horizontal]
R54  10k  R  [R_Axial_DIN0207_L6.3mm_D2.5mm_P7.62mm_Horizontal]
R55  10k  R  [R_Axial_DIN0207_L6.3mm_D2.5mm_P7.62mm_Horizontal]
R56  100  R  [R_Axial_DIN0207_L6.3mm_D2.5mm_P7.62mm_Horizontal]
R57  10k  R  [R_Axial_DIN0207_L6.3mm_D2.5mm_P7.62mm_Horizontal]
R58  10k  R  [R_Axial_DIN0207_L6.3mm_D2.5mm_P7.62mm_Horizontal]
R59  100  R  [R_Axial_DIN0207_L6.3mm_D2.5mm_P7.62mm_Horizontal]
R60  10k  R  [R_Axial_DIN0207_L6.3mm_D2.5mm_P7.62mm_Horizontal]
R61  10k  R  [R_Axial_DIN0207_L6.3mm_D2.5mm_P7.62mm_Horizontal]
RV18  200  POT  [Potentiometer_Bourns_3296W_Vertical]
RV19  200  POT  [Potentiometer_Bourns_3296W_Vertical]
RV20  200k  POT  [Potentiometer_Bourns_3296W_Vertical]
RV21  200k  POT  [Potentiometer_Bourns_3296W_Vertical]
RV22  10k  POT  [Potentiometer_Bourns_3296W_Vertical]
TP13  H7_BPF2  TP  [TestPoint_THTPad_D1.5mm_Drill0.7mm]
TP14  H7_AP2  TP  [TestPoint_THTPad_D1.5mm_Drill0.7mm]
TP15  H7_OUT  TP  [TestPoint_THTPad_D1.5mm_Drill0.7mm]
U13  TL082CP  TL082  [DIP-8_W7.62mm]
U14  TL082CP  TL082  [DIP-8_W7.62mm]
U15  TL082CP  TL082  [DIP-8_W7.62mm]

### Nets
GND: C26.2 C27.2 RV18.2 RV18.3 RV19.2 RV19.3 RV22.3 U13.3 U13.5 U15.3 ; also sheet 1,2,3,4,6
H7_AMPLITUDE: RV22.2 U15.5
H7_AP1: R55.1 R57.1 R59.1 U14.1
H7_AP2: J4.1 R58.1 R60.1 TP14.1 U14.7
H7_APINV1: R54.2 R55.2 U14.2
H7_APINV2: R57.2 R58.2 U14.6
H7_BPF1: C22.2 R50.1 R51.1 U13.1
H7_BPF2: C24.2 R53.1 R54.1 R56.1 TP13.1 U13.7
H7_INV1: C23.2 R50.2 U13.2
H7_INV2: C25.2 R53.2 U13.6
H7_LP1: C26.1 RV20.2 RV20.3 U14.3
H7_LP2: C27.1 RV21.2 RV21.3 U14.5
H7_NEG: J4.3 R61.1 U15.1
H7_NODE1: C22.1 C23.1 R48.2 R49.1
H7_NODE2: C24.1 C25.1 R51.2 R52.1
H7_OUT: TP15.1 U15.6 U15.7 ; also sheet 6
H7_PHR1: R56.2 RV20.1
H7_PHR2: R59.2 RV21.1
H7_POLINV: R60.2 R61.2 U15.2
H7_SELECT: J4.2 RV22.1
H7_TUNE1: R49.2 RV18.1
H7_TUNE2: R52.2 RV19.1
SQ: R48.1 ; also sheet 1,2,3,4
VCC: U13.8 U14.8 U15.8 ; also sheet 1,2,3,4,6
VEE: U13.4 U14.4 U15.4 ; also sheet 1,2,3,4,6

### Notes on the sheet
- Waveform synthesis: harmonic_7 (VCC=+12V, VEE=-12V)

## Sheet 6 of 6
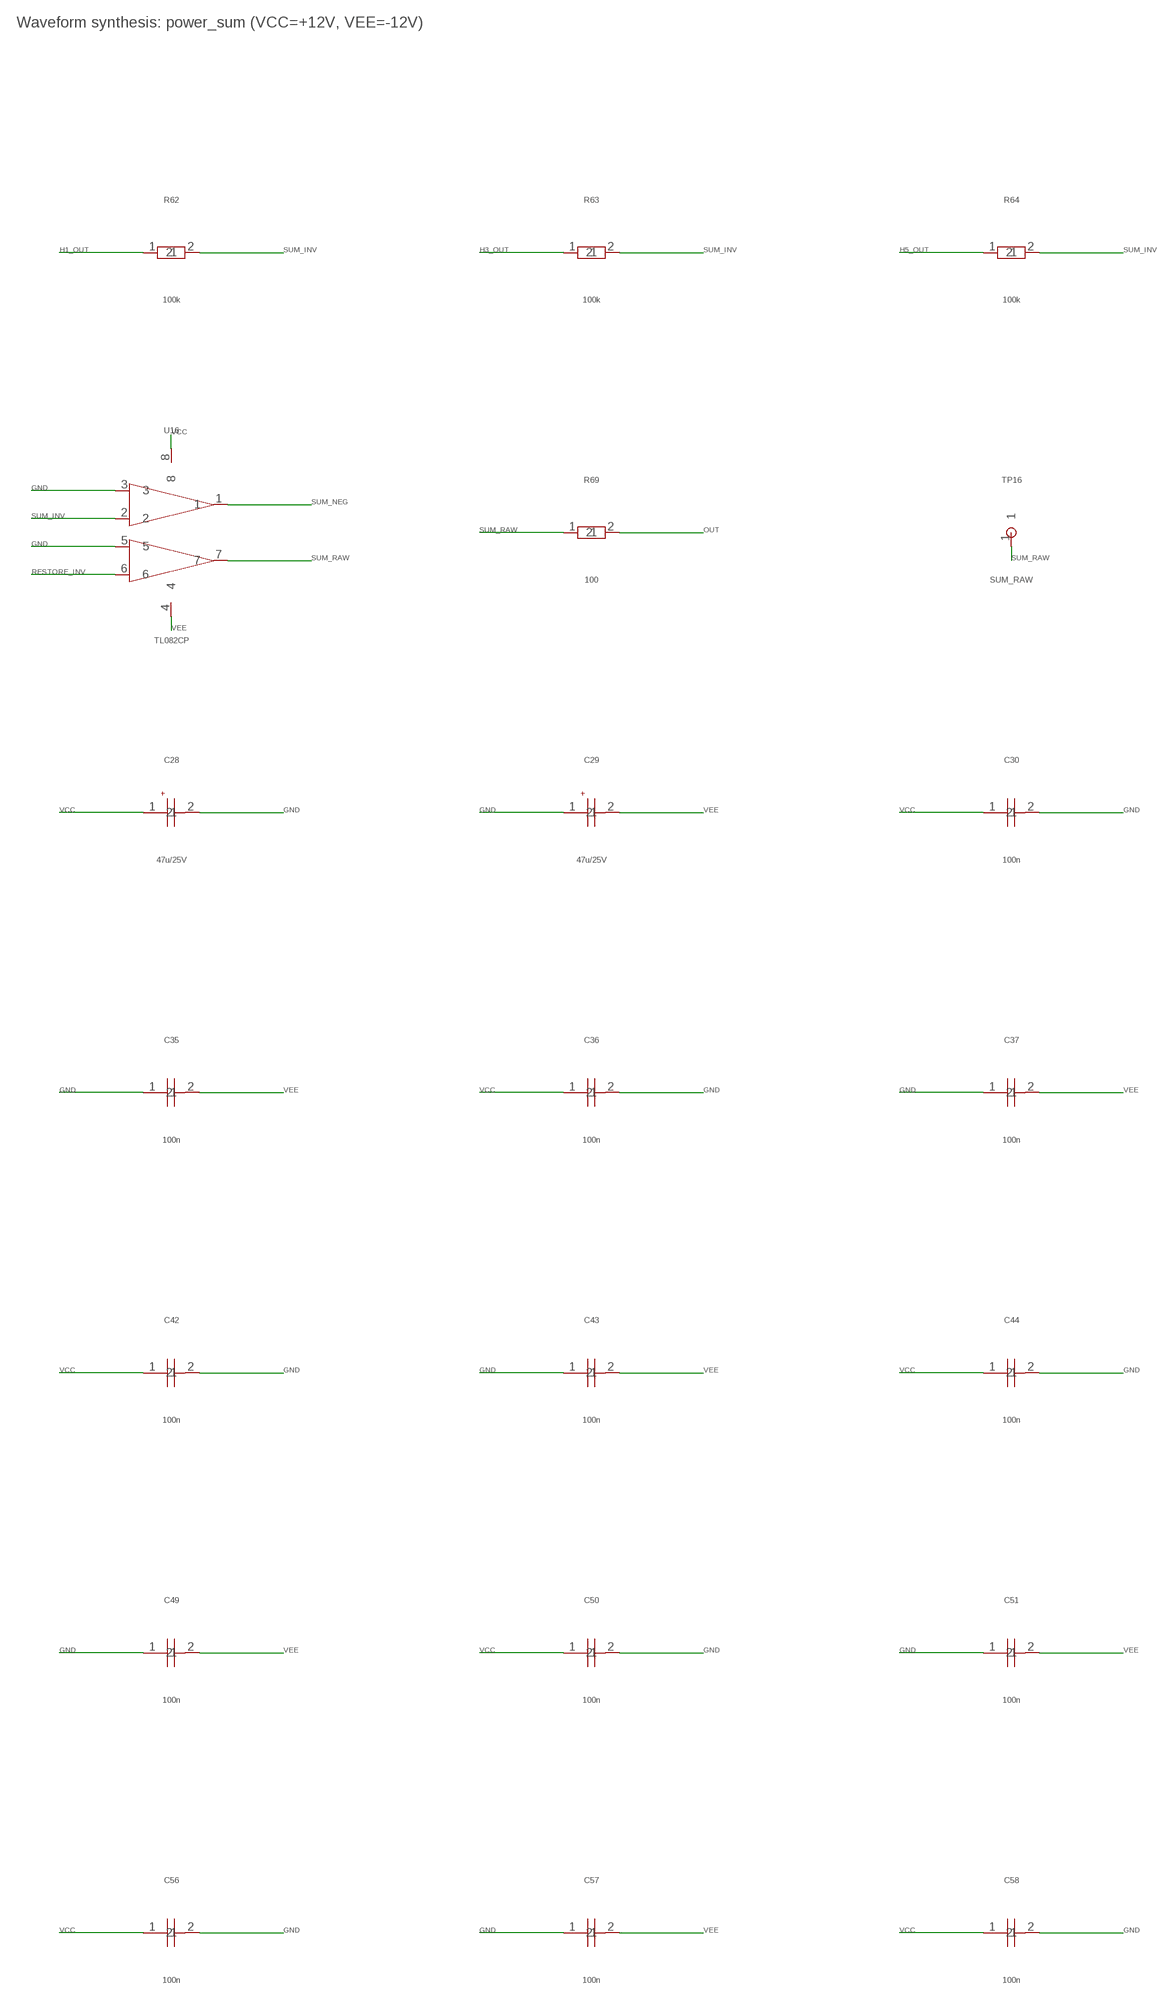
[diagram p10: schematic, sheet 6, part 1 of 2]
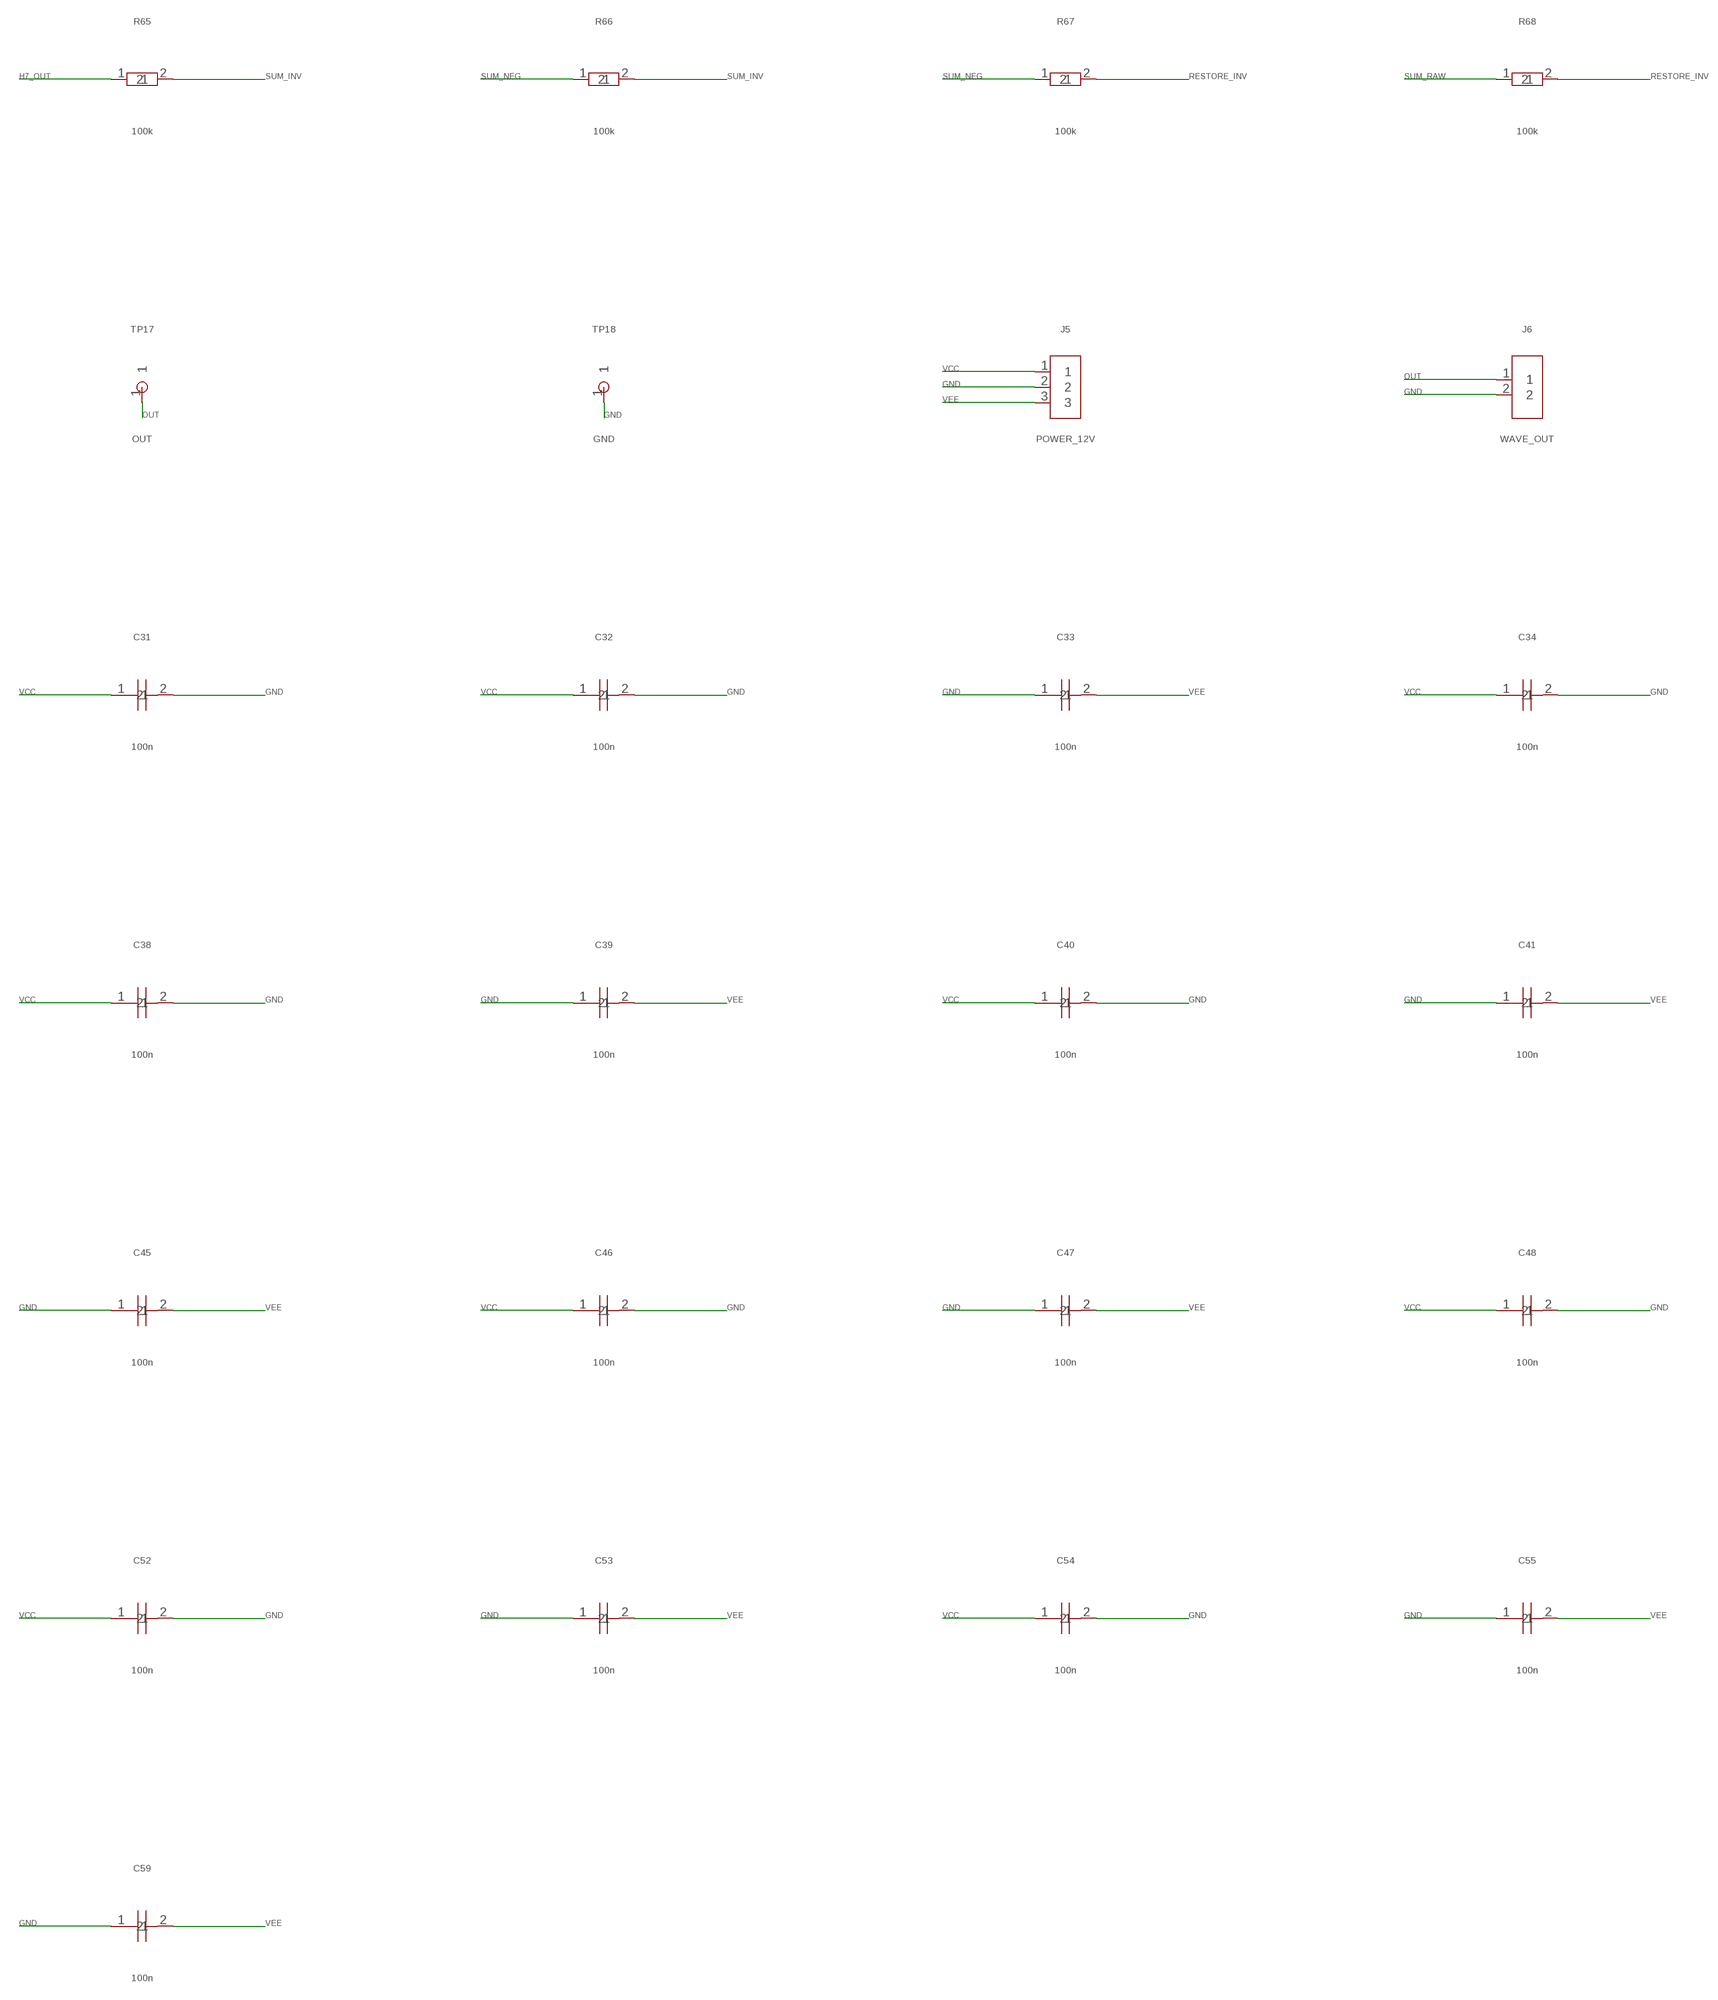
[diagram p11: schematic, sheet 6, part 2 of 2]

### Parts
C28  47u/25V  CP  [CP_Radial_D5.0mm_P2.00mm]
C29  47u/25V  CP  [CP_Radial_D5.0mm_P2.00mm]
C30  100n  C  [C_Disc_D5.0mm_W2.5mm_P5.00mm]
C31  100n  C  [C_Disc_D5.0mm_W2.5mm_P5.00mm]
C32  100n  C  [C_Disc_D5.0mm_W2.5mm_P5.00mm]
C33  100n  C  [C_Disc_D5.0mm_W2.5mm_P5.00mm]
C34  100n  C  [C_Disc_D5.0mm_W2.5mm_P5.00mm]
C35  100n  C  [C_Disc_D5.0mm_W2.5mm_P5.00mm]
C36  100n  C  [C_Disc_D5.0mm_W2.5mm_P5.00mm]
C37  100n  C  [C_Disc_D5.0mm_W2.5mm_P5.00mm]
C38  100n  C  [C_Disc_D5.0mm_W2.5mm_P5.00mm]
C39  100n  C  [C_Disc_D5.0mm_W2.5mm_P5.00mm]
C40  100n  C  [C_Disc_D5.0mm_W2.5mm_P5.00mm]
C41  100n  C  [C_Disc_D5.0mm_W2.5mm_P5.00mm]
C42  100n  C  [C_Disc_D5.0mm_W2.5mm_P5.00mm]
C43  100n  C  [C_Disc_D5.0mm_W2.5mm_P5.00mm]
C44  100n  C  [C_Disc_D5.0mm_W2.5mm_P5.00mm]
C45  100n  C  [C_Disc_D5.0mm_W2.5mm_P5.00mm]
C46  100n  C  [C_Disc_D5.0mm_W2.5mm_P5.00mm]
C47  100n  C  [C_Disc_D5.0mm_W2.5mm_P5.00mm]
C48  100n  C  [C_Disc_D5.0mm_W2.5mm_P5.00mm]
C49  100n  C  [C_Disc_D5.0mm_W2.5mm_P5.00mm]
C50  100n  C  [C_Disc_D5.0mm_W2.5mm_P5.00mm]
C51  100n  C  [C_Disc_D5.0mm_W2.5mm_P5.00mm]
C52  100n  C  [C_Disc_D5.0mm_W2.5mm_P5.00mm]
C53  100n  C  [C_Disc_D5.0mm_W2.5mm_P5.00mm]
C54  100n  C  [C_Disc_D5.0mm_W2.5mm_P5.00mm]
C55  100n  C  [C_Disc_D5.0mm_W2.5mm_P5.00mm]
C56  100n  C  [C_Disc_D5.0mm_W2.5mm_P5.00mm]
C57  100n  C  [C_Disc_D5.0mm_W2.5mm_P5.00mm]
C58  100n  C  [C_Disc_D5.0mm_W2.5mm_P5.00mm]
C59  100n  C  [C_Disc_D5.0mm_W2.5mm_P5.00mm]
J5  POWER_12V  CONN3  [PinHeader_1x03_P2.54mm_Vertical]
J6  WAVE_OUT  CONN2  [PinHeader_1x02_P2.54mm_Vertical]
R62  100k  R  [R_Axial_DIN0207_L6.3mm_D2.5mm_P7.62mm_Horizontal]
R63  100k  R  [R_Axial_DIN0207_L6.3mm_D2.5mm_P7.62mm_Horizontal]
R64  100k  R  [R_Axial_DIN0207_L6.3mm_D2.5mm_P7.62mm_Horizontal]
R65  100k  R  [R_Axial_DIN0207_L6.3mm_D2.5mm_P7.62mm_Horizontal]
R66  100k  R  [R_Axial_DIN0207_L6.3mm_D2.5mm_P7.62mm_Horizontal]
R67  100k  R  [R_Axial_DIN0207_L6.3mm_D2.5mm_P7.62mm_Horizontal]
R68  100k  R  [R_Axial_DIN0207_L6.3mm_D2.5mm_P7.62mm_Horizontal]
R69  100  R  [R_Axial_DIN0207_L6.3mm_D2.5mm_P7.62mm_Horizontal]
TP16  SUM_RAW  TP  [TestPoint_THTPad_D1.5mm_Drill0.7mm]
TP17  OUT  TP  [TestPoint_THTPad_D1.5mm_Drill0.7mm]
TP18  GND  TP  [TestPoint_THTPad_D1.5mm_Drill0.7mm]
U16  TL082CP  TL082  [DIP-8_W7.62mm]

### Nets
GND: C28.2 C29.1 C30.2 C31.2 C32.2 C33.1 C34.2 C35.1 C36.2 C37.1 C38.2 C39.1 C40.2 C41.1 C42.2 C43.1 C44.2 C45.1 C46.2 C47.1 C48.2 C49.1 C50.2 C51.1 C52.2 C53.1 C54.2 C55.1 C56.2 C57.1 C58.2 C59.1 J5.2 J6.2 TP18.1 U16.3 U16.5 ; also sheet 1,2,3,4,5
H1_OUT: R62.1 ; also sheet 2
H3_OUT: R63.1 ; also sheet 3
H5_OUT: R64.1 ; also sheet 4
H7_OUT: R65.1 ; also sheet 5
OUT: J6.1 R69.2 TP17.1
RESTORE_INV: R67.2 R68.2 U16.6
SUM_INV: R62.2 R63.2 R64.2 R65.2 R66.2 U16.2
SUM_NEG: R66.1 R67.1 U16.1
SUM_RAW: R68.1 R69.1 TP16.1 U16.7
VCC: C28.1 C30.1 C31.1 C32.1 C34.1 C36.1 C38.1 C40.1 C42.1 C44.1 C46.1 C48.1 C50.1 C52.1 C54.1 C56.1 C58.1 J5.1 U16.8 ; also sheet 1,2,3,4,5
VEE: C29.2 C33.2 C35.2 C37.2 C39.2 C41.2 C43.2 C45.2 C47.2 C49.2 C51.2 C53.2 C55.2 C57.2 C59.2 J5.3 U16.4 ; also sheet 1,2,3,4,5

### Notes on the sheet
- Waveform synthesis: power_sum (VCC=+12V, VEE=-12V)

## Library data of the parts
C1 C2 C4-C27 C30-C59 = Waveform:C
C3 C28 C29 = Waveform:CP
J1-J5 = Waveform:CONN3
J6 = Waveform:CONN2
R1-R69 = Waveform:R
RV1-RV22 = Waveform:POT
TP1-TP18 = Waveform:TP
U1 = Waveform:NE555
U2 = Waveform:4013
U3-U16 = Waveform:TL082

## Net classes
0 default: width 0.25 mm, drill 0.3 mm, clearance 0.2 mm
